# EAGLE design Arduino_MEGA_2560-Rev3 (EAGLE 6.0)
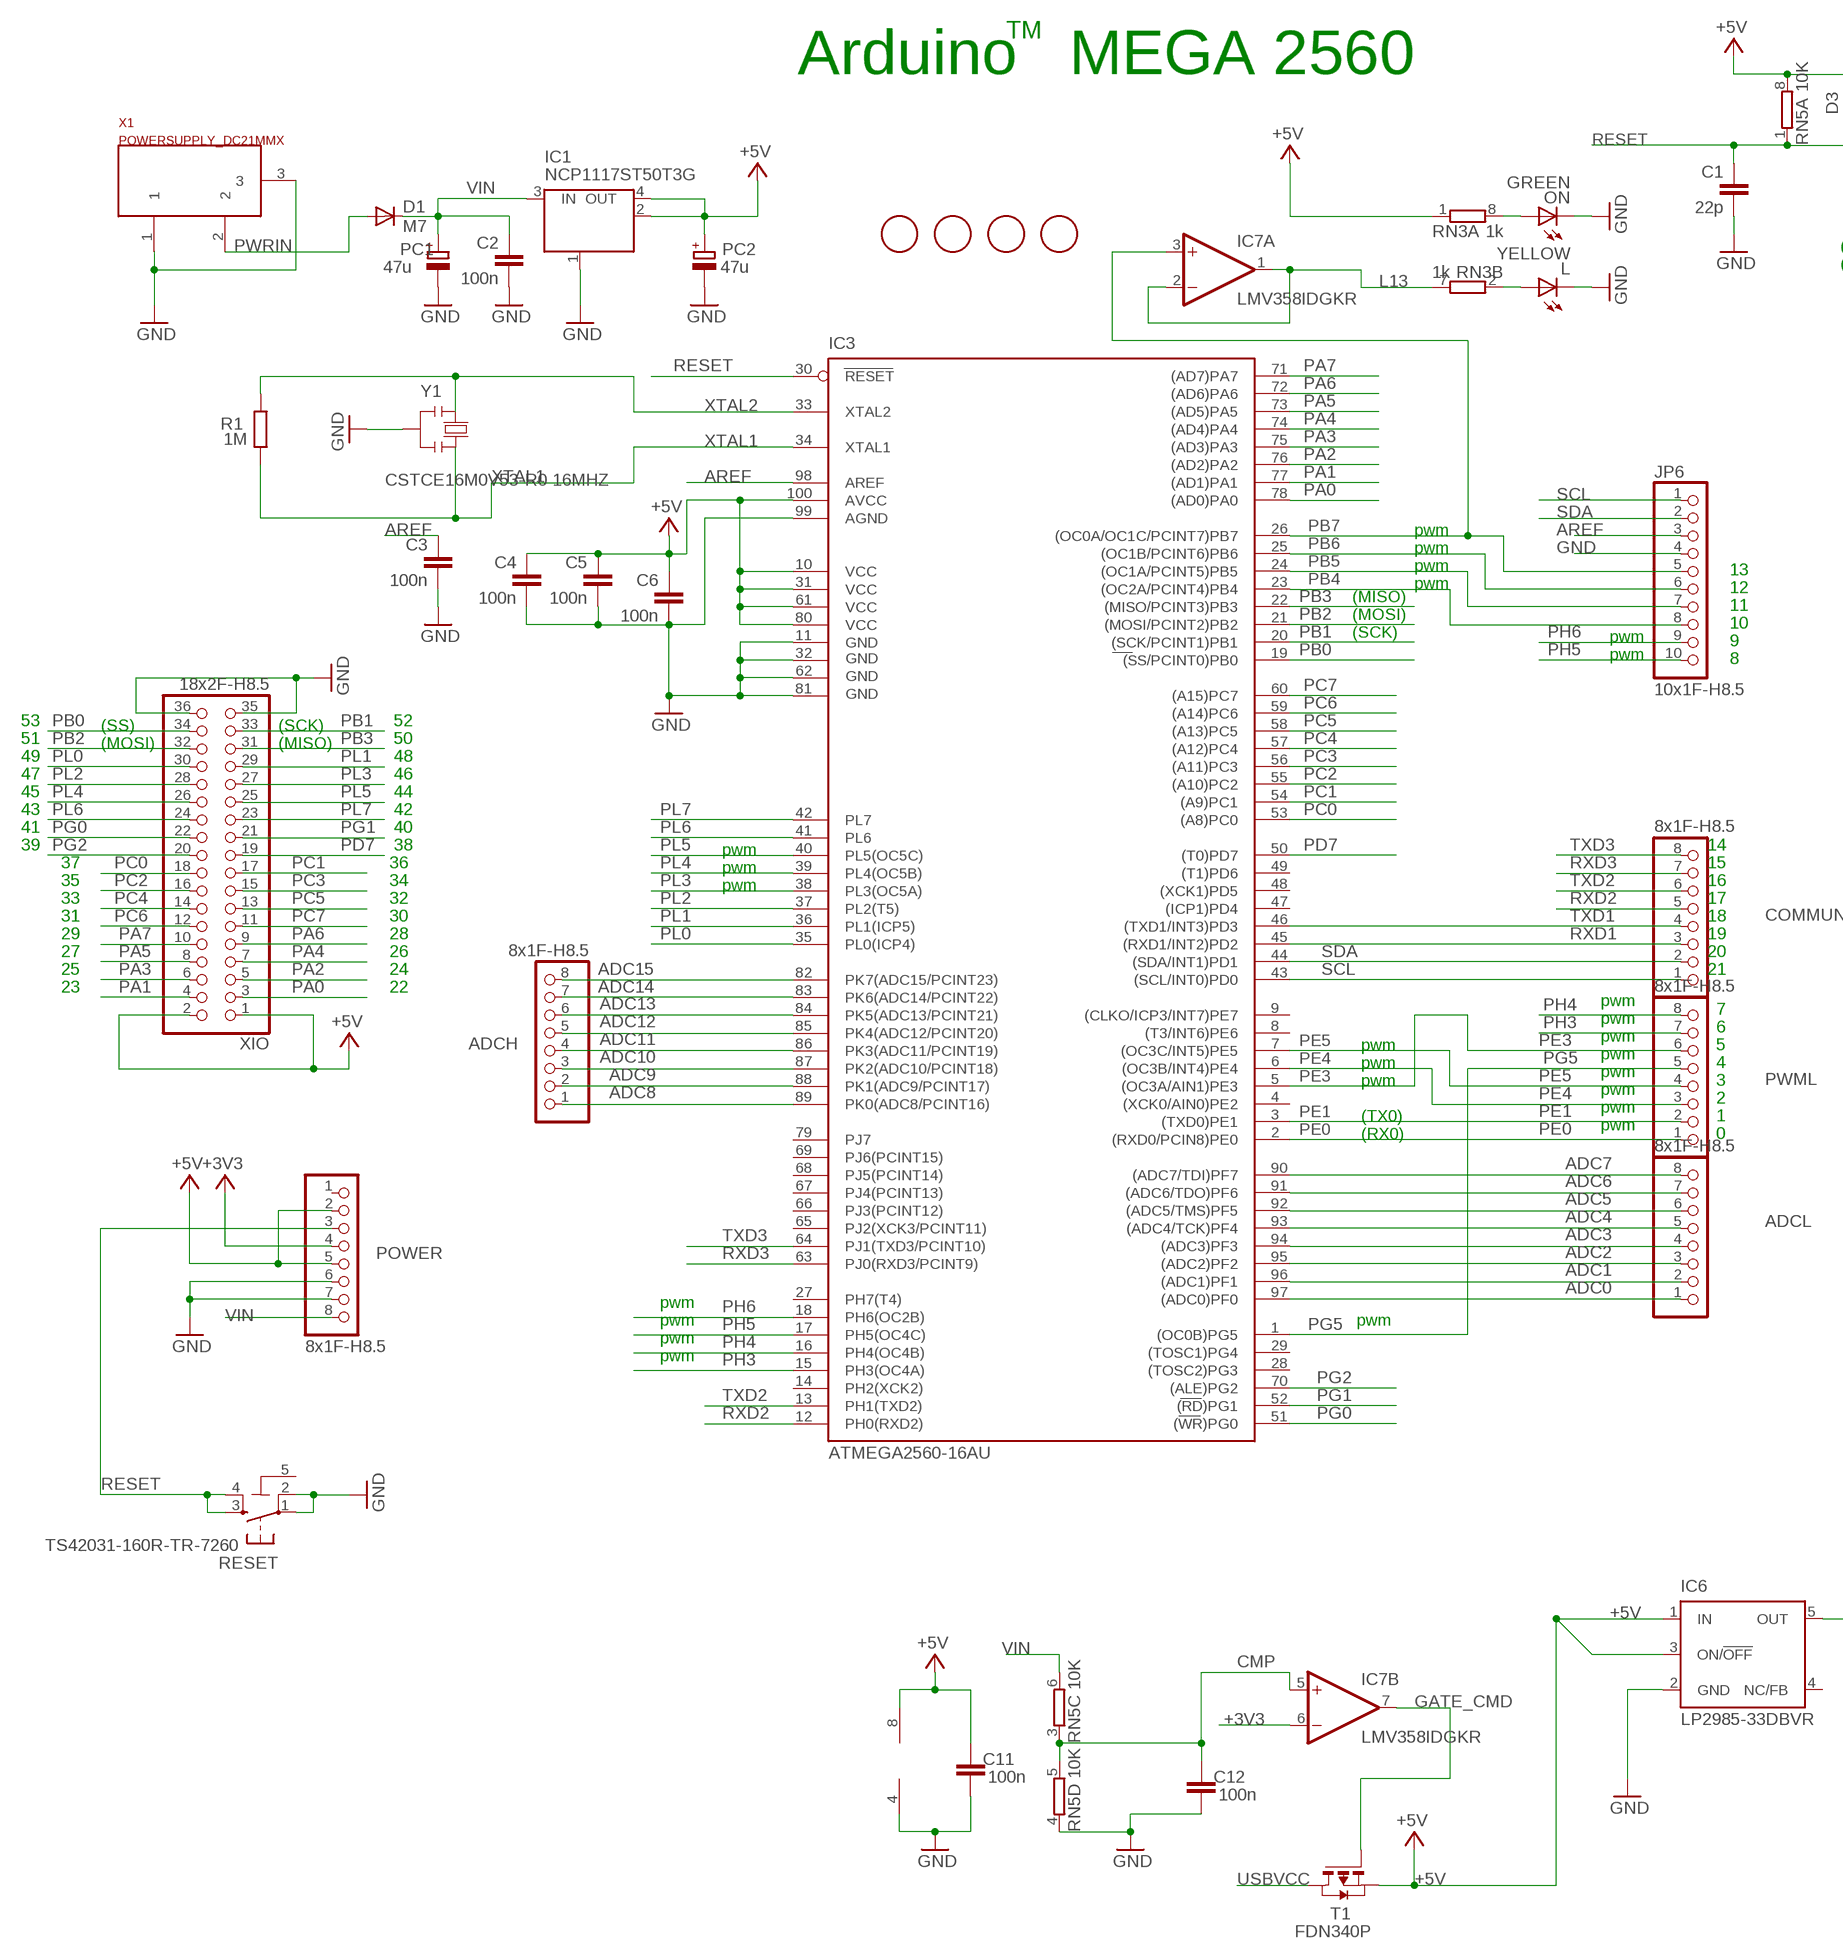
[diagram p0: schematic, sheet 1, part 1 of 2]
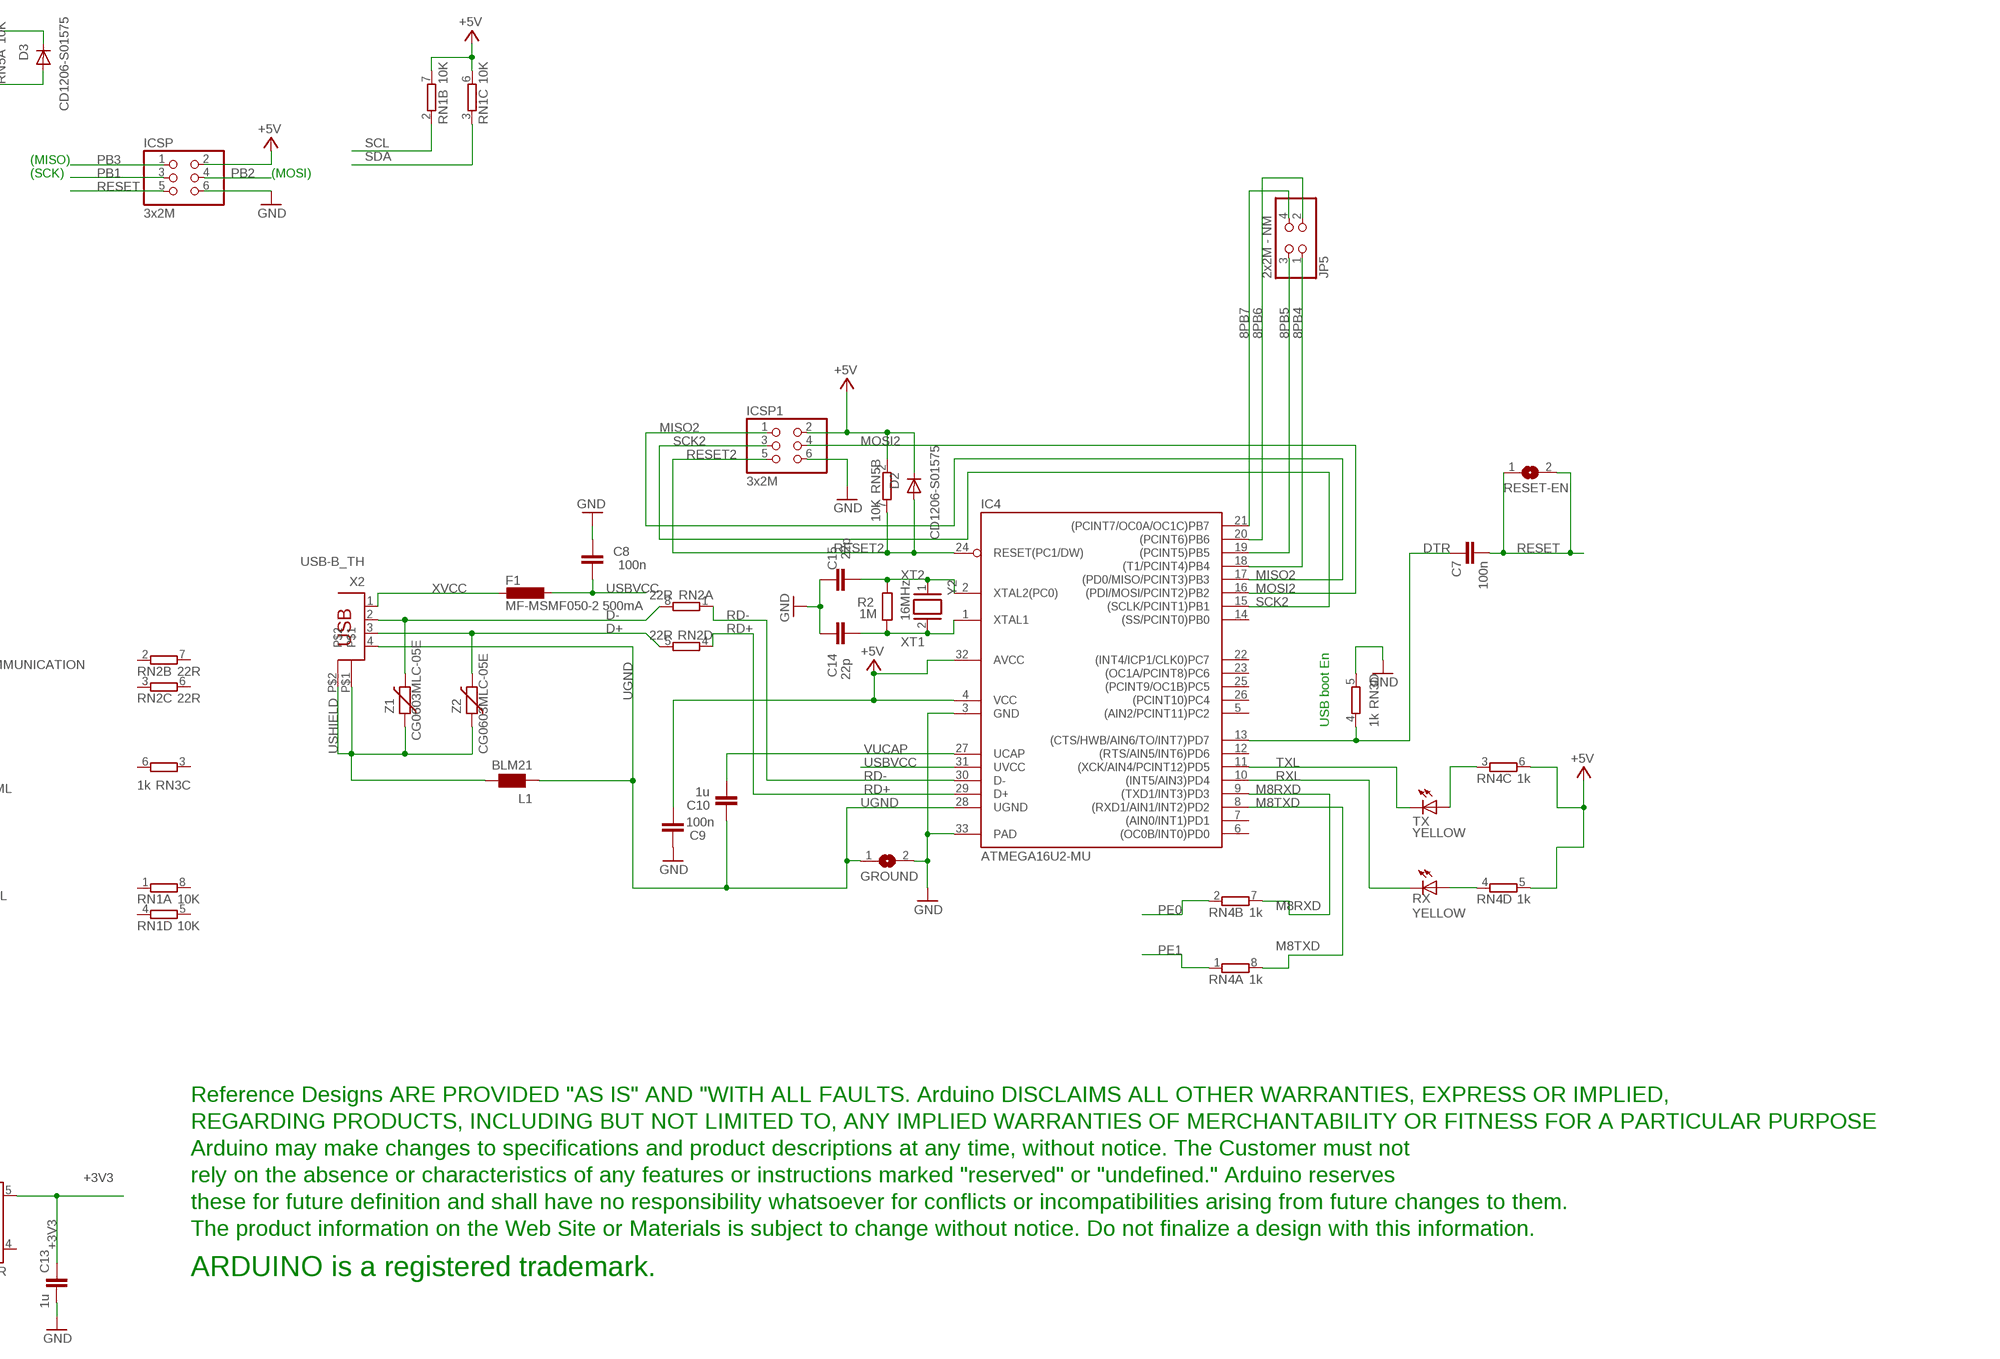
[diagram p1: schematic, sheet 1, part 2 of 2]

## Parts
ADCH  8x1F-H8.5  PINHD-1X8  [1X08]
ADCL  8x1F-H8.5  PINHD-1X8  [1X08]
C1  22p  C-EU0603-RND  [C0603-ROUND]
C2  100n  C-EU0603-RND  [C0603-ROUND]
C3  100n  C-EU0603-RND  [C0603-ROUND]
C4  100n  C-EU0603-RND  [C0603-ROUND]
C5  100n  C-EU0603-RND  [C0603-ROUND]
C6  100n  C-EU0603-RND  [C0603-ROUND]
C7  100n  C-EU0603-RND  [C0603-ROUND]
C8  100n  C-EU0603-RND  [C0603-ROUND]
C9  100n  C-EU0603-RND  [C0603-ROUND]
C10  1u  C-EU0603-RND  [C0603-ROUND]
C11  100n  C-EU0603-RND  [C0603-ROUND]
C12  100n  C-EU0603-RND  [C0603-ROUND]
C13  1u  C-EU0603-RND  [C0603-ROUND]
C14  22p  C-EU0603-RND  [C0603-ROUND]
C15  22p  C-EU0603-RND  [C0603-ROUND]
COMMUNICATION  8x1F-H8.5  PINHD-1X8  [1X08]
D1  M7  DIODE-SMB  [SMB]
D2  CD1206-S01575  DIODE-MINIMELF  [MINIMELF]
D3  CD1206-S01575  DIODE-MINIMELF  [MINIMELF]
F1  MF-MSMF050-2 500mA  L-EUL1812  [L1812]
FD1  FIDUCIALMOUNT  [FIDUCIA-MOUNT]
FD2  FIDUCIALMOUNT  [FIDUCIA-MOUNT]
FD3  FIDUCIALMOUNT  [FIDUCIA-MOUNT]
FD4  FIDUCIALMOUNT  [FIDUCIA-MOUNT]
GROUND  SJ  [SJ]
IC1  NCP1117ST50T3G  MC33269ST-3.3T3  [SOT223]
IC3  ATMEGA2560-16AU  ATMEGA25602560-16AU  [TQFP100]
IC4  ATMEGA16U2-MU  [MLF32]
IC6  LP2985-33DBVR  LP2985-XXDBVR33  [SOT23-DBV]
IC7  LMV358IDGKR  LMV358MMX  [MSOP08]
ICSP  3x2M  PINHD-2X3  [2X03]
ICSP1  3x2M  PINHD-2X3  [2X03]
JP5  2x2M - NM  PINHD-2X2  [2X02]
JP6  10x1F-H8.5  PINHD-1X10_ARD  [1X10]
L  YELLOW  LEDCHIP-LED0805  [CHIP-LED0805]
L1  BLM21  WE-CBF_0805  [0805]
ON  GREEN  LEDCHIP-LED0805  [CHIP-LED0805]
PC1  47u  CPOL-EUD  [PANASONIC_D]
PC2  47u  CPOL-EUD  [PANASONIC_D]
POWER  8x1F-H8.5  PINHD-1X8  [1X08]
PWML  8x1F-H8.5  PINHD-1X8  [1X08]
R1  1M  R-EU_R0603  [R0603-ROUND]
R2  1M  R-EU_R0603  [R0603-ROUND]
RESET  TS42031-160R-TR-7260  TS42  [TS42]
RESET-EN  SJ  [SJ]
RN1  10K  4R-NCAT16  [CAT16]
RN2  22R  4R-NCAY16  [CAY16]
RN3  1k  4R-NCAY16  [CAY16]
RN4  1k  4R-NCAY16  [CAY16]
RN5  10K  4R-NCAT16  [CAT16]
RX  YELLOW  LEDCHIP-LED0805  [CHIP-LED0805]
T1  FDN340P  PMOSSOT23  [SOT-23]
TX  YELLOW  LEDCHIP-LED0805  [CHIP-LED0805]
U$1  DISCLAIMER  [DISCLAIMER]
X1  POWERSUPPLY_DC21MMX  [POWERSUPPLY_DC-21MM]
X2  USB-B_TH  PN61729  [PN61729]
XIO  18x2F-H8.5  PINHD-2X18  [2X18]
Y1  CSTCE16M0V53-R0 16MHZ  RESONATORMU  [RESONATOR]
Y2  16MHz  XTAL/S  [QS]
Z1  CG0603MLC-05E  VARISTORCN0603  [CT/CN0603]
Z2  CG0603MLC-05E  VARISTORCN0603  [CT/CN0603]

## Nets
8PB4: IC4.18((T1/PCINT4)PB4) JP5.1
8PB5: IC4.19((PCINT5)PB5) JP5.3
8PB6: IC4.20((PCINT6)PB6) JP5.2
8PB7: IC4.21((PCINT7/OC0A/OC1C)PB7) JP5.4
+3V3 [power]: C13.2 IC6.5(OUT) IC7.6(B:-IN) POWER.4
+5V [power usb]: C4.1 C5.1 C6.1 C9.1 C11.2 D2.C D3.C IC1.2(OUT) IC1.4(OUT) IC3.10(VCC) IC3.31(VCC1) IC3.61(VCC2) IC3.80(VCC3) IC3.100(AVCC) IC4.4(VCC) IC4.32(AVCC) IC6.1(IN) IC6.3(ON/!OFF) IC7.8(P:V+) ICSP1.2 ICSP.2 PC2.+ POWER.2 POWER.5 RN1.6 RN1.7 RN3.1 RN4.5 RN4.6 RN5.2 RN5.8 T1.2(S) XIO.1 XIO.2
ADC0: ADCL.1 IC3.97((ADC0)PF0)
ADC1: ADCL.2 IC3.96((ADC1)PF1)
ADC2: ADCL.3 IC3.95((ADC2)PF2)
ADC3: ADCL.4 IC3.94((ADC3)PF3)
ADC4: ADCL.5 IC3.93((ADC4/TCK)PF4)
ADC5: ADCL.6 IC3.92((ADC5/TMS)PF5)
ADC6: ADCL.7 IC3.91((ADC6/TDO)PF6)
ADC7: ADCL.8 IC3.90((ADC7/TDI)PF7)
ADC8: ADCH.1 IC3.89(PK0(ADC8/PCINT16))
ADC9: ADCH.2 IC3.88(PK1(ADC9/PCINT17))
ADC10: ADCH.3 IC3.87(PK2(ADC10/PCINT18))
ADC11: ADCH.4 IC3.86(PK3(ADC11/PCINT19))
ADC12: ADCH.5 IC3.85(PK4(ADC12/PCINT20))
ADC13: ADCH.6 IC3.84(PK5(ADC13/PCINT21))
ADC14: ADCH.7 IC3.83(PK6(ADC14/PCINT22))
ADC15: ADCH.8 IC3.82(PK7(ADC15/PCINT23))
AREF: C3.1 IC3.98(AREF) JP6.3
CMP: C12.2 IC7.5(B:+IN) RN5.3 RN5.5
D+: RN2.5 X2.3 Z2.2
D-: RN2.8 X2.2 Z1.2
DTR: C7.1 IC4.13((CTS/HWB/AIN6/TO/INT7)PD7) RN3.4
GATE_CMD: IC7.7(B:OUT) T1.3(G)
GND [gnd]: C1.2 C2.2 C3.2 C4.2 C5.2 C6.2 C8.2 C9.2 C11.1 C12.1 C13.1 C14.2 C15.2 GROUND.2 IC1.1(GND/ADJ) IC3.11(GND) IC3.32(GND1) IC3.62(GND2) IC3.81(GND3) IC3.99(AGND) IC4.3(GND) IC4.33(PAD) IC6.2(GND) IC7.4(P:V-) ICSP1.6 ICSP.6 JP6.4 L.C ON.C PC1.- PC2.- POWER.6 POWER.7 RESET.1 RESET.2 RN3.5 RN5.4 X1.1 X1.3 XIO.35 XIO.36 Y1.2
L13: IC7.1(A:OUT) IC7.2(A:-IN) RN3.7
M8RXD: IC4.9((TXD1/INT3)PD3) RN4.7
M8TXD: IC4.8((RXD1/AIN1/INT2)PD2) RN4.8
MISO2: IC4.17((PD0/MISO/PCINT3)PB3) ICSP1.1
MOSI2: IC4.16((PDI/MOSI/PCINT2)PB2) ICSP1.4
N$2: L.A RN3.2
N$3: ON.A RN3.8
N$54: RN4.4 RX.A
N$55: RN4.3 TX.A
PA0: IC3.78((AD0)PA0) XIO.3
PA1: IC3.77((AD1)PA1) XIO.4
PA2: IC3.76((AD2)PA2) XIO.5
PA3: IC3.75((AD3)PA3) XIO.6
PA4: IC3.74((AD4)PA4) XIO.7
PA5: IC3.73((AD5)PA5) XIO.8
PA6: IC3.72((AD6)PA6) XIO.9
PA7: IC3.71((AD7)PA7) XIO.10
PB0: IC3.19((SS/PCINT0)PB0) XIO.34
PB1: IC3.20((SCK/PCINT1)PB1) ICSP.3 XIO.33
PB2: IC3.21((MOSI/PCINT2)PB2) ICSP.4 XIO.32
PB3: IC3.22((MISO/PCINT3)PB3) ICSP.1 XIO.31
PB4: IC3.23((OC2A/PCINT4)PB4) JP6.8
PB5: IC3.24((OC1A/PCINT5)PB5) JP6.7
PB6: IC3.25((OC1B/PCINT6)PB6) JP6.6
PB7: IC3.26((OC0A/OC1C/PCINT7)PB7) IC7.3(A:+IN) JP6.5
PC0: IC3.53((A8)PC0) XIO.18
PC1: IC3.54((A9)PC1) XIO.17
PC2: IC3.55((A10)PC2) XIO.16
PC3: IC3.56((A11)PC3) XIO.15
PC4: IC3.57((A12)PC4) XIO.14
PC5: IC3.58((A13)PC5) XIO.13
PC6: IC3.59((A14)PC6) XIO.12
PC7: IC3.60((A15)PC7) XIO.11
PD7: IC3.50((T0)PD7) XIO.19
PE0: IC3.2((RXD0/PCIN8)PE0) PWML.1 RN4.2
PE1: IC3.3((TXD0)PE1) PWML.2 RN4.1
PE3: IC3.5((OC3A/AIN1)PE3) PWML.6
PE4: IC3.6((OC3B/INT4)PE4) PWML.3
PE5: IC3.7((OC3C/INT5)PE5) PWML.4
PG0: IC3.51((WR)PG0) XIO.22
PG1: IC3.52((RD)PG1) XIO.21
PG2: IC3.70((ALE)PG2) XIO.20
PG5: IC3.1((OC0B)PG5) PWML.5
PH3: IC3.15(PH3(OC4A)) PWML.7
PH4: IC3.16(PH4(OC4B)) PWML.8
PH5: IC3.17(PH5(OC4C)) JP6.10
PH6: IC3.18(PH6(OC2B)) JP6.9
PL0: IC3.35(PL0(ICP4)) XIO.30
PL1: IC3.36(PL1(ICP5)) XIO.29
PL2: IC3.37(PL2(T5)) XIO.28
PL3: IC3.38(PL3(OC5A)) XIO.27
PL4: IC3.39(PL4(OC5B)) XIO.26
PL5: IC3.40(PL5(OC5C)) XIO.25
PL6: IC3.41(PL6) XIO.24
PL7: IC3.42(PL7) XIO.23
PWRIN [power]: D1.A X1.2
RD+: IC4.29(D+) RN2.4
RD-: IC4.30(D-) RN2.1
RESET: C1.1 C7.2 D3.A IC3.30(RESET) ICSP.5 POWER.3 RESET-EN.1 RESET-EN.2 RESET.3 RESET.4 RN5.1
RESET2: D2.A IC4.24(RESET(PC1/DW)) ICSP1.5 RN5.7
RXD1: COMMUNICATION.3 IC3.45((RXD1/INT2)PD2)
RXD2: COMMUNICATION.5 IC3.12(PH0(RXD2))
RXD3: COMMUNICATION.7 IC3.63(PJ0(RXD3/PCINT9))
RXL: IC4.10((INT5/AIN3)PD4) RX.C
SCK2: IC4.15((SCLK/PCINT1)PB1) ICSP1.3
SCL: COMMUNICATION.1 IC3.43((SCL/INT0)PD0) JP6.1 RN1.2
SDA: COMMUNICATION.2 IC3.44((SDA/INT1)PD1) JP6.2 RN1.3
TXD1: COMMUNICATION.4 IC3.46((TXD1/INT3)PD3)
TXD2: COMMUNICATION.6 IC3.13(PH1(TXD2))
TXD3: COMMUNICATION.8 IC3.64(PJ1(TXD3/PCINT10))
TXL: IC4.11((XCK/AIN4/PCINT12)PD5) TX.C
UGND [gnd]: C10.2 GROUND.1 IC4.28(UGND) L1.1 X2.4
USBVCC [power usb]: C8.1 F1.1 IC4.31(UVCC) T1.1(D)
USHIELD [gnd]: L1.2 X2.P$1 X2.P$2 Z1.1 Z2.1
VIN [power]: C2.1 D1.C IC1.3(IN) PC1.+ POWER.8 RN5.6
VUCAP: C10.1 IC4.27(UCAP)
XT1: C14.1 IC4.1(XTAL1) R2.1 Y2.2
XT2: C15.1 IC4.2(XTAL2(PC0)) R2.2 Y2.1
XTAL1: IC3.34(XTAL1) R1.1 Y1.3
XTAL2: IC3.33(XTAL2) R1.2 Y1.1
XVCC [power usb]: F1.2 X2.1
Unconnected: IC3.4((XCK0/AIN0)PE2) IC3.8((T3/INT6)PE6) IC3.9((CLKO/ICP3/INT7)PE7) IC3.14(PH2(XCK2)) IC3.27(PH7(T4)) IC3.28((TOSC2)PG3) IC3.29((TOSC1)PG4) IC3.47((ICP1)PD4) IC3.48((XCK1)PD5) IC3.49((T1)PD6) IC3.65(PJ2(XCK3/PCINT11)) IC3.66(PJ3(PCINT12)) IC3.67(PJ4(PCINT13)) IC3.68(PJ5(PCINT14)) IC3.69(PJ6(PCINT15)) IC3.79(PJ7) IC4.5((AIN2/PCINT11)PC2) IC4.6((OC0B/INT0)PD0) IC4.7((AIN0/INT1)PD1) IC4.12((RTS/AIN5/INT6)PD6) IC4.14((SS/PCINT0)PB0) IC4.22((INT4/ICP1/CLK0)PC7) IC4.23((OC1A/PCINT8)PC6) IC4.25((PCINT9/OC1B)PC5) IC4.26((PCINT10)PC4) IC6.4(NC/FB) POWER.1 RN1.1 RN1.4 RN1.5 RN1.8 RN2.2 RN2.3 RN2.6 RN2.7 RN3.3 RN3.6

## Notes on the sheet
- TM
- Arduino   MEGA 2560
- (MISO)
- (SCK) | (MOSI)
- pwm
- pwm
- pwm | 13
- pwm | 12
- (MISO)
- 11
- (MOSI)
- 10
- (SCK) | pwm
- 9
- pwm | 8
- 53 | (SS) | (SCK) | 52
- 51 | (MOSI) | (MISO) | 50
- 49 | 48
- 47 | 46
- 45 | 44
- 43 | 42
- 41 | 40
- 39 | 38 | pwm | 14
- 37 | 36 | pwm | 15
- 35 | 34 | pwm | 16
- 33 | 32 | 17
- 31 | 30 | 18
- 29 | 28 | 19
- 27 | 26 | 20
- 25 | 24 | 21
- 23 | 22 | USB boot En
- pwm
- 7
- pwm
- 6
- pwm
- pwm | 5
- pwm
- pwm | 4
- pwm
- pwm | 3
- pwm
- 2
- pwm
- (TX0) | 1
- pwm
- (RX0) | 0
- pwm
- pwm | pwm
- pwm
- pwm

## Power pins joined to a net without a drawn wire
5-GND: RESET.5(5-GND)

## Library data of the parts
ADCH ADCL COMMUNICATION POWER PWML = SmartPrj:PINHD-1X8: PIN HEADER
C1-C15 = SmartPrj:C-EU: CAPACITOR, European symbol
D1-D3 = diode:DIODE-: DIODE
F1 = rcl:L-EU: INDUCTOR, European symbol
FD1-FD4 = SmartPrj:FIDUCIALMOUNT
GROUND RESET-EN = jumper:SJ: SMD solder JUMPER
IC1 = linear:MC33269ST*: Adjustable Output Low Dropout Voltage Regulator 800 mA Source: http://www.onsemi.com/pub/Collateral/MC33269-D.PDF
IC3 = SmartPrj:ATMEGA2560: MICROCONTROLLER 64/128/256 Kbytes FLASH 4 Kbytes EEPROM 8 Kbytes SRAM 86 General Purpose I/O pins 12-channels16-bit PWM 4 x Serial USARTs 16-channels 10-bit A/D
IC4 = SmartPrj:ATMEGA16U2-
IC6 = SmartPrj:LP2985-XXDBVR: ULTRALOW-POWER 50-mA LOW-DROPOUT LINEAR REGULATORS 50-mA Low-Dropout Regulator Source: http://focus.ti.com/lit/ds/symlink/tps77001.pdf
IC7 = linear:LMV358?*: Dual General Purpose, Low Voltage, Rail-to-Rail Output Operational Amplifiers Source: http://www.national.com/mpf/LM/LMV321.html http://www.national.com/dt/lmv_qual.pdf
ICSP ICSP1 = SmartPrj:PINHD-2X3: PIN HEADER
JP5 = SmartPrj:PINHD-2X2: PIN HEADER
JP6 = SmartPrj:PINHD-1X10_ARD: PIN HEADER
L ON RX TX = led:LED: LED
L1 = wuerth-elektronik:WE-CBF: SMD EMI Suppression Ferrite Beads
PC1 PC2 = rcl:CPOL-EU: POLARIZED CAPACITOR, European symbol
R1 R2 = SmartPrj:R-EU_: RESISTOR, European symbol
RESET = SmartPrj:TS42: TS42 Dongnan Electronics Tact switch VDC 12V - 50mA
RN1-RN5 = resistor-dil:4R-N: Array Chip Resistor Source: RS Component / Phycomp
T1 = zetex:PMOSSOT23: MOS FET
U$1 = SmartPrj:DISCLAIMER
X1 = SmartPrj:POWERSUPPLY_DC21MM
X2 = SmartPrj:PN61729: BERG USB connector
XIO = SmartPrj:PINHD-2X18: PIN HEADER
Y1 = SmartPrj:RESONATOR
Y2 = SmartPrj:XTAL/S: CRYSTAL
Z1 Z2 = varistor:VARISTOR: VARISTOR

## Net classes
0 default: width 0.203 mm, drill 0.406 mm, clearance 0.203 mm
1 power: width 0.61 mm, drill 0.406 mm, clearance 0.203 mm
2 gnd: width 0.305 mm, drill 0.406 mm, clearance 0.203 mm
3 power usb: width 0.508 mm, drill 0.406 mm, clearance 0.203 mm

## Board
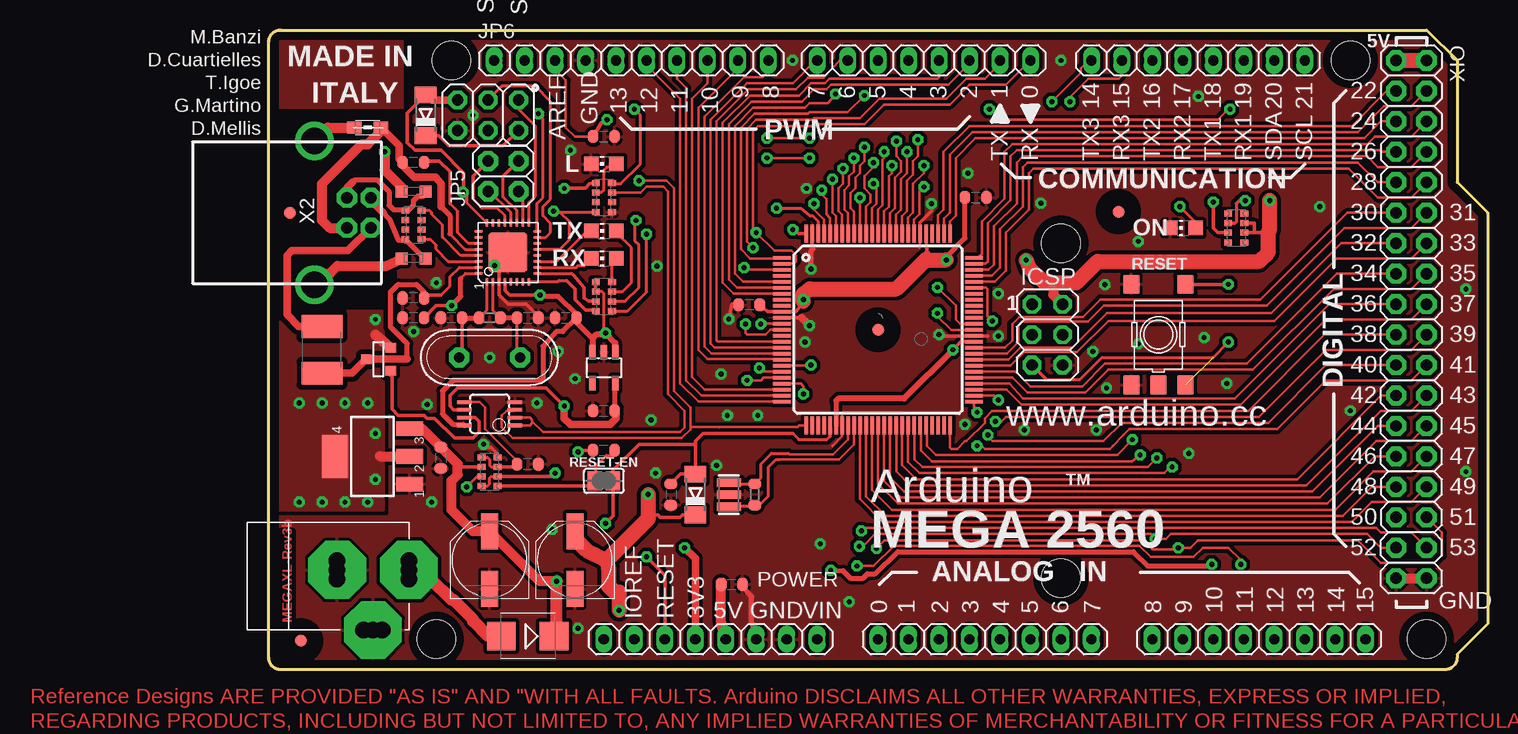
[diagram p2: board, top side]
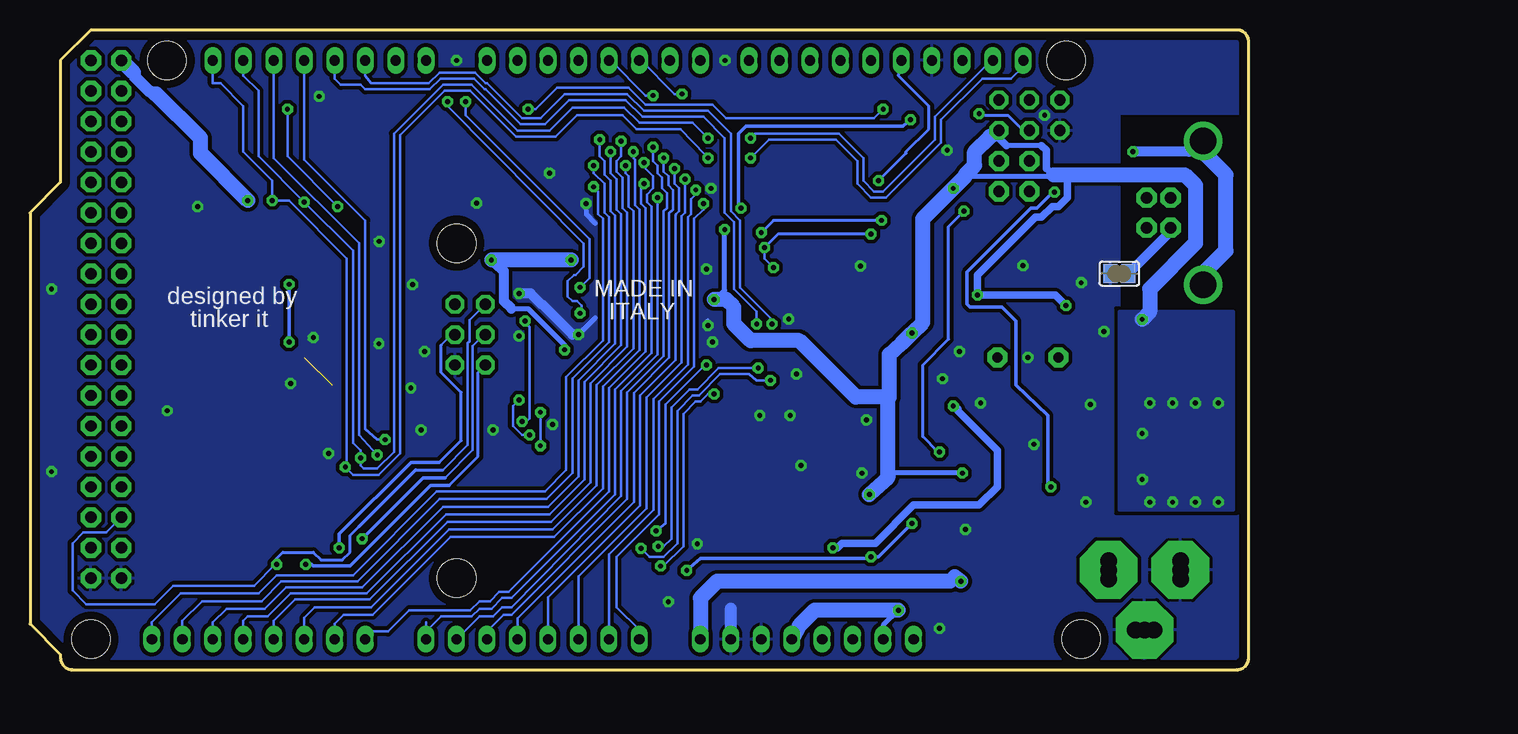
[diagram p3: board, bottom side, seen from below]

Size 101.6 x 53.34 mm. Coordinates in mm from the lower left corner, seen from the top.
Outline: 96.52,53.34 99.06,50.8 99.06,40.64 101.6,38.1 101.6,3.81 99.06,1.27 99.06,1 arc-90 98.06,0 1,0 arc-90 0,1 0,52.34 arc-90 1,53.34 96.52,53.34
Copper layers (1*16): Top 0.035mm / dielectric 1.5mm / Bottom 0.035mm
Design rules: minimum track width 8mil, minimum drill 16mil, track to track 7mil, track to pad 7mil, pad to pad 8mil, via to via 10mil, smd to smd 7mil, copper to edge 27mil, drill to drill 12mil, minimum pad ring 10mil, minimum via ring 10mil, stop-mask expansion 2mil, vias tented up to drill 24mil, thermal gap 10mil
Holes 3.2 mm at 96.52,2.54 15.24,50.8 90.17,50.8 13.97,2.54 66.04,35.56 66.04,7.62

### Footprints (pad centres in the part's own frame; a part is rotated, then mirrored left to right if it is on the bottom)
1X08 = drill 0.85 pad 1.422 long: 1 -8.89,0; 2 -6.35,0; 3 -3.81,0; 4 -1.27,0; 5 1.27,0; 6 3.81,0; 7 6.35,0; 8 8.89,0
C0603-ROUND = smd 0.898 x 1.1: 1 -0.889,0; 2 0.889,0
SMB = smd 2.4 x 2.4: A 2.2,0; C -2.2,0
MINIMELF = smd 1.4 x 1.8: A 1.7,0; C -1.7,0
L1812 = smd 1.9 x 3.4: 1 -1.95,0; 2 1.95,0
FIDUCIA-MOUNT = smd 1.016 x 1.016: P$1 0,0
SJ = smd 1.168 x 1.6: 1 -0.762,0; 2 0.762,0
SOT223 = smd 1.219 x 2.235: 1 -2.311,-3.099; 2 0,-3.099; 3 2.311,-3.099 | smd 3.6 x 2.2: 4 0,3.099
TQFP100 = smd 1.5 x 0.3: 1 -8,6; 2 -8,5.5; 3 -8,5; 4 -8,4.5; 5 -8,4; 6 -8,3.5; 7 -8,3; 8 -8,2.5; 9 -8,2; 10 -8,1.5; 11 -8,1; 12 -8,0.5; 13 -8,0; 14 -8,-0.5; 15 -8,-1; 16 -8,-1.5; 17 -8,-2; 18 -8,-2.5; 19 -8,-3; 20 -8,-3.5; 21 -8,-4; 22 -8,-4.5; 23 -8,-5; 24 -8,-5.5; 25 -8,-6; 51 8,-6; 52 8,-5.5; 53 8,-5; 54 8,-4.5; 55 8,-4; 56 8,-3.5; 57 8,-3; 58 8,-2.5; 59 8,-2; 60 8,-1.5; 61 8,-1; 62 8,-0.5; 63 8,0; 64 8,0.5; 65 8,1; 66 8,1.5; 67 8,2; 68 8,2.5; 69 8,3; 70 8,3.5; 71 8,4; 72 8,4.5; 73 8,5; 74 8,5.5; 75 8,6 | smd 0.3 x 1.5: 26 -6,-8; 27 -5.5,-8; 28 -5,-8; 29 -4.5,-8; 30 -4,-8; 31 -3.5,-8; 32 -3,-8; 33 -2.5,-8; 34 -2,-8; 35 -1.5,-8; 36 -1,-8; 37 -0.5,-8; 38 0,-8; 39 0.5,-8; 40 1,-8; 41 1.5,-8; 42 2,-8; 43 2.5,-8; 44 3,-8; 45 3.5,-8; 46 4,-8; 47 4.5,-8; 48 5,-8; 49 5.5,-8; 50 6,-8; 76 6,8; 77 5.5,8; 78 5,8; 79 4.5,8; 80 4,8; 81 3.5,8; 82 3,8; 83 2.5,8; 84 2,8; 85 1.5,8; 86 1,8; 87 0.5,8; 88 0,8; 89 -0.5,8; 90 -1,8; 91 -1.5,8; 92 -2,8; 93 -2.5,8; 94 -3,8; 95 -3.5,8; 96 -4,8; 97 -4.5,8; 98 -5,8; 99 -5.5,8; 100 -6,8
MLF32 = smd 0.7 x 0.28: 1 -2.45,1.75; 2 -2.45,1.25; 3 -2.45,0.75; 4 -2.45,0.25; 5 -2.45,-0.25; 6 -2.45,-0.75; 7 -2.45,-1.25; 8 -2.45,-1.75; 17 2.45,-1.75; 18 2.45,-1.25; 19 2.45,-0.75; 20 2.45,-0.25; 21 2.45,0.25; 22 2.45,0.75; 23 2.45,1.25; 24 2.45,1.75 | smd 0.28 x 0.7: 9 -1.75,-2.45; 10 -1.25,-2.45; 11 -0.75,-2.45; 12 -0.25,-2.45; 13 0.25,-2.45; 14 0.75,-2.45; 15 1.25,-2.45; 16 1.75,-2.45; 25 1.75,2.45; 26 1.25,2.45; 27 0.75,2.45; 28 0.25,2.45; 29 -0.25,2.45; 30 -0.75,2.45; 31 -1.25,2.45; 32 -1.75,2.45 | smd 3.254 x 3.254: 33 0,0
SOT23-DBV = smd 0.55 x 1.2: 1 -0.95,-1.3; 2 0,-1.3; 3 0.95,-1.3; 4 0.95,1.3; 5 -0.95,1.3
MSOP08 = smd 0.3 x 1.2: 1 -0.976,-2.113; 2 -0.326,-2.113; 3 0.324,-2.113; 4 0.974,-2.113; 5 0.974,2.112; 6 0.324,2.112; 7 -0.326,2.112; 8 -0.976,2.112
2X03 = drill 0.95 pad 1.55 octagon: 1 -2.54,-1.27; 2 -2.54,1.27; 3 0,-1.27; 4 0,1.27; 5 2.54,-1.27; 6 2.54,1.27
2X02 = drill 0.95 pad 1.676 octagon: 1 -1.27,-1.27; 2 -1.27,1.27; 3 1.27,-1.27; 4 1.27,1.27
1X10 = drill 0.85 pad 1.422 long: 1 -11.43,0; 2 -8.89,0; 3 -6.35,0; 4 -3.81,0; 5 -1.27,0; 6 1.27,0; 7 3.81,0; 8 6.35,0; 9 8.89,0; 10 11.43,0
CHIP-LED0805 = smd 1.2 x 1.2: A 0,-1.05; C 0,1.05
0805 = smd 1.2 x 1: 1 -1.1,0; 2 1.1,0
PANASONIC_D = smd 3 x 1.4: + 2.4,0; - -2.4,0
R0603-ROUND = smd 0.898 x 1.1: 1 -0.889,0; 2 0.889,0
TS42 = smd 1.6 x 1.4: 1 -4.2,2.25; 2 4.2,2.25; 3 -4.2,-2.25; 4 4.2,-2.25; 5 -4.2,0
CAT16 = smd 0.5 x 0.65: 1 -1.2,-0.675; 2 -0.4,-0.675; 3 0.4,-0.675; 4 1.2,-0.675; 5 1.2,0.675; 6 0.4,0.675; 7 -0.4,0.675; 8 -1.2,0.675
CAY16 = smd 0.5 x 0.65: 1 -1.2,-0.675; 2 -0.4,-0.675; 3 0.4,-0.675; 4 1.2,-0.675; 5 1.2,0.675; 6 0.4,0.675; 7 -0.4,0.675; 8 -1.2,0.675
SOT-23 = smd 0.787 x 0.889: 1 0.025,-1.016; 2 -0.94,1.016; 3 0.991,1.016
POWERSUPPLY_DC-21MM = drill 1.4 pad 4.826 octagon: 1 -5.08,-3.353; 2 -0.076,-6.35; 3 -0.076,-0.356 | drill 1.4: 4 -5.08,-4.115; 5 -5.08,-2.591; 6 -0.838,-0.356; 7 0.686,-0.356; 8 -0.838,-6.35; 9 0.686,-6.35
PN61729 = drill 0.95 pad 1.676 octagon: 1 1.25,4.71; 2 -1.25,4.71; 3 -1.25,2.71; 4 1.25,2.71 | drill 2.2: P$1 -6,0; P$2 6,0
2X18 = drill 0.95 pad 1.676 octagon: 1 -21.59,-1.27; 2 -21.59,1.27; 3 -19.05,-1.27; 4 -19.05,1.27; 5 -16.51,-1.27; 6 -16.51,1.27; 7 -13.97,-1.27; 8 -13.97,1.27; 9 -11.43,-1.27; 10 -11.43,1.27; 11 -8.89,-1.27; 12 -8.89,1.27; 13 -6.35,-1.27; 14 -6.35,1.27; 15 -3.81,-1.27; 16 -3.81,1.27; 17 -1.27,-1.27; 18 -1.27,1.27; 19 1.27,-1.27; 20 1.27,1.27; 21 3.81,-1.27; 22 3.81,1.27; 23 6.35,-1.27; 24 6.35,1.27; 25 8.89,-1.27; 26 8.89,1.27; 27 11.43,-1.27; 28 11.43,1.27; 29 13.97,-1.27; 30 13.97,1.27; 31 16.51,-1.27; 32 16.51,1.27; 33 19.05,-1.27; 34 19.05,1.27; 35 21.59,-1.27; 36 21.59,1.27
RESONATOR = smd 0.7 x 2: 1 -1,0; 2 0,0; 3 1,0
QS = drill 0.85 pad 1.676 octagon: 1 -2.54,0; 2 2.54,0
CT/CN0603 = smd 1 x 1: 1 -1,0; 2 1,0

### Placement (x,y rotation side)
ADCH  82.55,2.54 0 top
ADCL  59.69,2.54 0 top
C1  33.53,14.61 270 top
C2  14.35,17.65 270 top
C3  27.94,44.45 0 top
C4  38.61,7.11 0 top
C5  58.93,39.37 0 top
C6  40.05,30.42 180 top
C7  27.94,18.29 0 top
C8  12.06,30.99 180 top
C9  12.06,29.34 180 top
C10  12.06,42.29 180 top
C11  24.77,29.34 0 top
C12  21.59,17.14 180 top
C13  27.94,21.59 0 top
C14  15.24,29.34 180 top
C15  21.59,29.34 0 top
COMMUNICATION  77.47,50.8 180 top
D1  21.59,2.79 180 top
D2  13.08,46.23 90 top
D3  35.56,14.61 90 top
F1  4.45,26.67 90 top
FD1  70.84,38.19 0 top
FD2  2.67,2.41 0 top
FD3  1.78,38.1 0 top
FD4  50.8,28.35 0 top
GROUND  10.79,33.02 180 bottom
IC1  8.64,17.78 90 top
IC3  50.8,28.35 0 top
IC4  19.94,34.8 90 top
IC6  27.94,25.17 180 top
IC7  18.41,21.34 90 top
ICSP  64.9,27.94 270 top
ICSP1  18.29,46.23 180 top
JP5  19.56,41.15 90 top
JP6  30.23,50.8 0 top
L  27.94,42.16 90 top
L1  8.26,45.21 180 top
ON  76.2,36.83 90 top
PC1  18.41,9.14 90 top
PC2  25.53,9.14 90 top
POWER  36.83,2.54 0 top
PWML  54.61,50.8 180 top
R1  40.51,14.61 90 top
R2  18.41,29.34 0 top
RESET  74.17,27.94 90 top
RESET-EN  27.94,15.75 0 top
RN1  80.64,36.83 270 top
RN2  12.06,37.08 90 top
RN3  27.94,39.37 270 top
RN4  27.94,31.11 90 top
RN5  18.41,16.51 90 top
RX  27.94,34.29 90 top
T1  9.14,25.91 270 top
TX  27.94,36.58 90 top
U$1  not placed on the board
X1  5.33,8.38 90 top
X2  3.81,38.1 270 top
XIO  95.25,29.21 270 top
Y1  38.35,14.61 270 top
Y2  18.41,26.04 180 top
Z1  12.06,34.29 0 top
Z2  12.06,39.88 0 top

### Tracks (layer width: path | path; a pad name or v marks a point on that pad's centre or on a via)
8PB4
  Top 0.254: 20.57,39.88 JP5.1 21.19,39.52 IC4.18
8PB5
  Top 0.254: 19.56,41.15 19.56,39.42 20.69,38.29 IC4.19
  Top 0.305: 19.56,41.15 JP5.3
8PB6
  Top 0.254: IC4.20 20.19,38.1 18.41,39.88 JP5.2
8PB7
  Top 0.254: IC4.21 19.68,37.85 19.05,38.48 17.78,38.48 17.02,39.24 17.02,39.37
  Top 0.305: 17.02,39.37 17.02,41.15 JP5.4
+3V3  (via drill 0.41)
  Top 0.305: IC7.6 15.42,21.66 15.11,21.97 15.11,22.86 15.75,23.5 23.11,23.5 v24.64,21.97
  Top 0.406: 28.89,21.62 IC6.5
  Top 0.61: POWER.4 35.56,9.27 v34.67,10.16 | 28.89,21.62 C13.2 28.96,21.55 28.96,20.95 28.45,20.45 25.15,20.45 24.64,20.95 v24.64,21.97
  Bottom 0.61: v34.67,10.16 34.29,10.16 33.91,10.54 31.11,10.54 27.94,13.72 22.48,13.72 20.95,15.24 20.95,18.29 24.26,21.59 24.26,21.72 v24.64,21.97
+5V  (via drill 0.41)
  Top 0.254: IC3.80 54.81,36.3 54.79,36.27 54.81,36.25 54.81,35.41 | 57.66,27.3 57.7,27.35 | v28.07,28.07 28,28.19 27.94,28.64 27.94,31.37 27.79,31.52 RN4.6 RN4.5 | RN5.8 18.23,15.31 18.41,15.49 18.41,16 18.52,16.11 RN5.2 | IC4.32 16.41,33.05 16,32.64
  Top 0.305: 54.86,34.67 54.86,35.1 54.81,35.15 54.81,35.41 | 57.7,27.35 IC3.61 | v57.02,26.67 57.66,27.3 | 44.45,30.48 43.94,29.85 IC3.10 41.59,29.85 C6.1 | IC3.100 44.17,36.35 v43.69,36.7 | 83.31,36.45 82.17,36.45 | v24.64,40.13 26.42,40.13 26.74,40.51 RN3.1 | RN1.6 82.15,36.43 82.17,36.45 | 82.17,36.45 82.17,37.21 82.15,37.23 RN1.7 | C9.1 13.97,30.35 v15.24,30.35 | RN5.2 23.6,16.11 v23.88,16.38 | IC4.4 19.69,31.62 20.07,31.24 v22.61,31.24 | D2.C 14.15,44.53 14.99,43.69 19.56,43.69 ICSP1.2 | D3.C 34.49,12.9 34.29,12.7 32.64,12.7 32.43,12.9 31.93,12.9 31.62,13.21
  Top 0.406: 44.55,30.7 44.45,30.48 v44.58,30.86 | 47.3,22.41 IC3.31 | C5.1 58.04,35.97 56.52,34.42 56.49,34.39 v56.49,34.16 | C11.2 25.53,29.09 26.99,27.62 | C11.2 25.65,29.59 24.13,31.11 22.73,31.11 v22.61,31.24 | C11.2 24.51,28.19 23.96,28.19 22.86,26.96 22.86,24.26 22.61,24.13 15.37,24.13 14.48,23.24 14.48,21.34 15.37,20.45 16.22,20.45 IC7.8 | 16,32.64 16,31.11 v15.24,30.35
  Top 0.508: 47.3,22.41 47.5,22.61 52.96,22.61 v57.02,26.67 | 26.96,26.67 IC6.3 26.99,27.62 27.3,27.94 27.94,27.94 | IC6.1 28.89,27.24 v28.07,28.07
  Top 0.61: v28.07,28.07 27.94,27.94 | 54.86,34.67 54.86,34.29 54.99,34.16
  Top 0.813: 9.27,17.78 IC1.2 | C4.1 37.72,3.94 POWER.5 | 83.31,34.8 83.31,34.92 | 65.41,32.26 65.41,31.24 ICSP.2 | T1.2 10.11,26.85 8.89,27.94
  Top 1.27: XIO.1 XIO.2 | v63.14,34.14 63.37,33.53 64.64,32.26 65.41,32.26 67.31,32.26 69.09,34.04 82.55,34.04 83.31,34.8 | 83.31,34.92 83.31,36.45 83.44,36.7 v83.44,39.12 | 44.55,30.7 44.55,31.34 45.09,31.75 52.32,31.75 54.74,34.16 54.99,34.16 v56.49,34.16 | v31.62,14.61 31.62,13.21 31.62,12.57 28.13,9.08 | v29.21,4.95 29.21,6.48 28.83,6.48 28.32,6.99 28.32,8.51 28.13,9.08 | PC2.+ 25.53,10.92 26.54,9.91 27.05,9.65 28.13,9.08
  Bottom 0.406: v44.58,30.86 44.58,30.73 43.69,31.62 v43.69,36.7 | 61.47,30.1 60.07,30.1 57.02,27.05 v57.02,26.67 | 23.5,41.15 16.76,41.15 16.64,41.27 16.26,41.27 | 17.27,43.69 20.19,43.69 | v23.88,16.38 30.1,16.38 | POWER.2 30.48,3.68 v29.21,4.95
  Bottom 0.61: 63.12,34.16 v63.14,34.14 | 23.62,41.27 23.5,41.15 | 16.26,41.27 16.89,41.78 16.89,43.31 17.27,43.69 | 20.19,43.69 20.83,44.32 ICSP1.2 | v15.24,30.35 16.13,31.24 v22.61,31.24 22.61,32.89 17.78,37.72 17.27,37.72 16.38,38.61 15.88,38.61 15.11,39.37 15.11,41.27
  Bottom 0.813: 61.47,30.1 62.1,30.73 62.1,33.27 v63.14,34.14
  Bottom 1.016: 91.19,48.01 91.69,48.26 92.84,49.4 92.96,49.78
  Bottom 1.27: v29.21,4.95 36.2,4.95 37.47,3.68 POWER.5 | v56.49,34.16 63.12,34.16 | v44.58,30.86 43.56,30.86 42.93,30.23 42.93,28.83 41.53,27.43 37.47,27.43 32.77,22.73 30.1,22.73 | ICSP1.2 20.95,44.83 21.59,44.45 22.86,43.18 22.86,42.04 23.62,41.27 23.62,41.15 v24.64,40.13 27.18,37.59 27.18,28.96 v28.07,28.07 28.96,27.18 29.97,26.29 29.97,22.73 30.1,22.73 | 30.1,22.73 30.1,16.38 30.1,16 v31.62,14.61 | v83.44,39.12 87.38,43.05 87.38,44.32 91.06,48.01 91.19,48.01 | v8.89,29.21 8.26,29.84 8.26,31.75 4.45,35.56 4.45,40.39 5.33,41.27 15.11,41.27 16.26,41.27 | 92.96,49.78 XIO.1
  other vias: 6.35,22.23 4.45,22.23 8.26,22.23 2.54,22.23 8.89,19.68 2.54,13.97 6.35,13.97 4.45,13.97 8.89,15.88 8.26,13.97
  pour Top (isolate 0.406, no thermals): 9.53,13.34 9.53,29.84 0.64,29.84 0.64,13.34
  pour Bottom: 1.27,13.34 1.27,29.84 10.79,29.84 10.79,13.34
ADC0  (via drill 0.41)
  Top 0.203: IC3.97 46.3,37.52 45.47,38.35 v45.47,38.86
  Bottom 0.203: ADCL.1 50.8,3.3 52.7,5.21 52.7,9.4 49.15,12.95 49.15,22.35 46.23,25.27 46.23,37.59 45.47,38.35 v45.47,38.86
ADC1  (via drill 0.41)
  Top 0.203: IC3.96 46.8,37.66 46.48,37.97 46.48,39.24 46.1,39.62 v46.1,40.01
  Bottom 0.203: ADCL.2 53.34,9.6 49.63,13.31 49.63,22.55 46.74,25.45 46.74,37.72 46.48,37.97 46.48,39.24 46.1,39.62 v46.1,40.01
ADC2  (via drill 0.41)
  Top 0.203: v46.99,40.89 46.99,38.1 47.27,37.82 47.27,36.68 47.37,36.58 47.3,36.51 47.3,36.38 47.27,36.35 | 47.27,36.35 47.24,36.32 | 47.27,36.35 IC3.95
  Bottom 0.203: ADCL.3 55.88,7.8 50.22,13.46 50.22,22.68 47.27,25.63 47.27,37.82 46.99,38.1 v46.99,40.89
ADC3  (via drill 0.41)
  Top 0.203: IC3.94 47.8,37.92 47.5,38.23 47.5,40.13 47.88,40.51 v47.88,41.78
  Bottom 0.203: ADCL.4 58.42,2.74 58.52,2.85 58.52,3.05 58.42,3.15 58.42,6.02 50.75,13.69 50.75,22.86 47.8,25.81 47.8,37.85 47.75,37.97 47.5,38.23 47.5,40.13 47.88,40.51 v47.88,41.78
ADC4  (via drill 0.41)
  Top 0.203: IC3.93 48.3,38.06 48.01,38.35 48.01,40.01 48.39,40.39 48.39,41.15 48.77,41.53 v48.77,42.67
  Bottom 0.203: 60.96,2.44 ADCL.5 60.96,4.27 51.26,13.97 51.26,23.06 48.31,26.01 48.31,38.05 48.01,38.35 48.01,40.01 48.39,40.39 48.39,41.15 48.77,41.53 v48.77,42.67
ADC5  (via drill 0.41)
  Top 0.203: IC3.92 48.8,38.2 48.51,38.48 48.51,39.75 48.9,40.13 48.9,41.02 49.28,41.4 49.28,42.04 49.66,42.42 v49.66,43.56
  Bottom 0.203: v49.66,43.56 49.66,42.42 49.28,42.04 49.28,41.4 48.9,41.02 48.9,40.13 48.51,39.75 48.51,38.48 48.77,38.23 48.77,26.16 51.82,23.11 51.82,14.22 61.47,4.57 62.1,4.57 63.5,3.17 ADCL.6
ADC6  (via drill 0.41)
  Top 0.203: IC3.91 49.3,39.35 v49.28,39.37
  Bottom 0.203: v49.28,39.37 49.28,26.29 52.32,23.24 52.32,14.48 61.47,5.21 62.23,5.21 62.99,4.45 64.14,4.45 ADCL.7
ADC7  (via drill 0.41)
  Top 0.203: IC3.90 49.8,38.62 50.16,38.99 50.16,39.62 49.66,40.13 49.66,41.15 50.42,41.91 v50.42,42.29
  Bottom 0.203: v50.42,42.29 50.42,41.91 49.66,41.15 49.66,40.13 50.16,39.62 50.16,38.99 49.78,38.61 49.78,26.42 52.83,23.37 52.83,14.61 61.47,5.97 62.23,5.97 63.12,5.08 64.14,5.08 64.77,4.45 67.31,4.45 68.58,3.17 | 68.58,3.17 ADCL.8 | 68.58,3.17 68.58,3.94
ADC8  (via drill 0.41)
  Top 0.203: IC3.89 50.3,38.49 50.67,38.86 50.67,40.26 v50.42,40.51
  Bottom 0.203: v50.42,40.51 50.67,40.26 50.67,38.86 50.29,38.48 50.29,26.54 53.34,23.5 53.34,14.86 61.72,6.48 62.48,6.48 63.25,5.71 64.14,5.71 64.9,4.95 69.98,4.95 71.75,3.17 73.66,3.17 ADCH.1
ADC9  (via drill 0.41)
  Top 0.203: IC3.88 50.8,38.35 51.18,38.73 51.18,42.55 51.31,42.67 v51.31,43.18
  Bottom 0.203: v51.31,43.18 51.31,42.67 51.18,42.55 51.18,38.73 50.8,38.35 50.8,26.67 53.85,23.62 53.85,15.11 57.91,11.05 66.55,11.05 73.03,4.57 75.44,4.57 76.2,3.81 ADCH.2
ADC10  (via drill 0.41)
  Top 0.203: IC3.87 51.3,38.22 51.69,38.61 51.69,41.15 51.94,41.4 v51.94,42.04
  Bottom 0.203: v51.94,42.04 51.94,41.4 51.69,41.15 51.69,38.61 51.31,38.23 51.31,26.8 54.36,23.75 54.36,15.37 58.04,11.68 66.67,11.68 73.15,5.21 77.85,5.21 78.74,4.32 ADCH.3
ADC11  (via drill 0.41)
  Top 0.203: IC3.86 51.8,38.08 52.2,38.48 52.2,41.02 52.7,41.53 52.7,42.42 52.32,42.8 v52.32,44.07
  Bottom 0.203: v52.32,44.07 52.32,42.8 52.7,42.42 52.7,41.53 52.2,41.02 52.2,38.48 51.82,38.1 51.82,26.92 54.86,23.88 54.86,15.62 58.17,12.32 66.8,12.32 73.28,5.84 79.5,5.84 81.28,4.06 ADCH.4
ADC12  (via drill 0.41)
  Top 0.203: IC3.85 52.3,37.95 52.7,38.35 52.7,40.89 53.21,41.4 v53.21,43.18
  Bottom 0.203: v53.21,43.18 53.21,41.4 52.7,40.89 52.7,38.35 52.32,37.97 52.32,27.05 55.37,24 55.37,15.88 58.29,12.95 66.93,12.95 73.53,6.35 79.88,6.35 81.79,4.45 83.44,4.45 83.82,4.06 ADCH.5
ADC13  (via drill 0.41)
  Top 0.203: IC3.84 52.8,37.81 53.21,38.23 53.21,40.77 53.72,41.27 53.72,42.42 54.1,42.8 v54.1,44.2
  Bottom 0.203: v54.1,44.2 54.1,42.8 53.72,42.42 53.72,41.27 53.21,40.77 53.21,38.23 52.83,37.85 52.83,27.18 55.88,24.13 55.88,16.13 58.42,13.59 67.18,13.59 73.91,6.86 80.26,6.86 82.04,5.08 85.22,5.08 86.36,3.94 ADCH.6
ADC14  (via drill 0.41)
  Top 0.203: IC3.83 53.3,37.68 53.72,38.1 53.72,40.51 54.61,41.4 v54.61,42.04
  Bottom 0.203: v54.61,42.04 54.61,41.4 53.72,40.51 53.72,38.1 53.34,37.72 53.34,27.3 56.39,24.26 56.39,16.38 58.55,14.22 67.44,14.22 74.3,7.37 80.64,7.37 82.3,5.71 87.25,5.71 88.9,4.06 ADCH.7
ADC15  (via drill 0.41)
  Top 0.203: IC3.82 53.8,37.54 54.23,37.97 54.23,39.88 v54.61,40.26
  Bottom 0.203: v54.61,40.26 54.23,39.88 54.23,37.97 53.85,37.59 53.85,27.43 56.9,24.38 56.9,16.64 58.67,14.86 67.69,14.86 74.68,7.87 81.03,7.87 82.55,6.35 89.03,6.35 91.44,3.94 ADCH.8
AREF  (via drill 0.41)
  Top 0.203: C3.1 25.53,44.45 24.77,45.21 24.77,49.15 23.88,50.04 JP6.3
  Top 0.254: IC3.98 45.8,37.38 45.34,37.85 45.09,37.85 44.32,38.48 v42.34,38.48
  Top 0.305: v28.19,45.85 27.73,45.59 C3.1
  Bottom 0.305: v28.19,45.85 28.83,45.34 41.91,45.34 42.55,44.7 42.55,38.66 v42.34,38.48
CMP
  Top 0.203: C12.2 20.7,17.4 18.03,20.07 18.03,21.84 17.57,22.31 IC7.5
  Top 0.254: 19.07,16.89 18.54,16.89 18.41,17.02 18.41,17.53 18.23,17.71 RN5.5
  Top 0.305: 19.07,16.89 RN5.3 | RN5.3 19.87,16.91 | C12.2 20.47,16.91 RN5.3
D+
  Top 0.406: 6.99,40.64 7.2,40.85 9.06,40.85 10.03,39.88 10.03,38.73 10.41,38.35 11.32,38.35 RN2.5 11.61,38.28 12.06,38.73 12.06,39.12 12.45,39.5 12.94,39.5 Z2.2
  Top 0.61: X2.3 6.52,40.17 6.99,40.64
D-
  Top 0.406: 9.53,38.1 9.56,38.1 10.03,37.63 10.03,37.59 10.79,35.81 11.32,35.81 RN2.8 12.73,34.54 Z1.2
  Top 0.61: X2.2 8.53,39.1 9.53,38.1
DTR  (via drill 0.41)
  Top 0.254: 24.26,38.17 23.81,38.17 v23.75,38.23 | 24.26,38.17 RN3.4 | IC4.13 24.25,35.05 25.02,35.81 25.02,37.41 24.26,38.17
  Top 0.305: C7.1 26.04,18.29 v25.78,18.16
  Bottom 0.254: v25.78,18.16 25.91,18.16 27.18,19.43 27.18,25.4 25.02,27.56 25.02,36.96 v23.75,38.23
GATE_CMD
  Top 0.305: T1.3 10.29,24.79 10.29,21.72 10.79,21.21 12.95,21.21 13.21,20.95 13.84,20.95 15.49,19.3 17.02,19.3 17.53,19.81 17.53,20.7 17.22,21.01 IC7.7
  Top 0.406: T1.3 10.16,24.64
GND  (via drill 0.41)
  Top 0.203: 54.23,35.18 54.3,35.25 IC3.81 54.33,36.35 | 54.3,37.28 54.3,36.38 54.33,36.35 | IC3.32 47.8,21.39 47.88,21.46 52.83,21.46 | IC3.32 | IC3.32 47.8,19.48 46.99,18.67 | 54.33,36.35 54.36,36.32
  Top 0.305: IC1.1 11.81,15.49 | 45.39,35.1 45.29,35.2 IC3.99 | IC3.11 42.86,29.35 42.88,29.36 44.32,29.36 | 44.32,29.36 44.4,29.36 | 56.06,27.86 56.08,27.84 58.81,27.84 | 58.83,27.84 58.82,27.85 IC3.62 58.81,27.84 | 54.3,37.28 55.24,38.23 v55.24,38.86 | 44.32,29.36 44.32,29.34 44.35,29.36 44.42,29.36 | v38.35,29.23 38.61,30.48 | 59.94,27.81 59.92,27.84 58.81,27.84 | v18.82,33.68 19.23,33.68 | C15.2 22.48,29.46 21.46,30.48 19.94,30.48 19.19,31.23 IC4.3 | IC4.33 19.94,33.33 v18.82,33.68 | v18.82,33.68 19.19,33.31 | 19.19,32.33 19.19,33.33 v18.82,33.68 | RN5.4 19.09,17.99 18.54,18.54 18.16,18.54 v17.91,18.8
  Top 0.406: C4.2 39.88,6.48 40.26,6.1 40.26,3.94 POWER.6 | 56.06,27.86 56.01,27.81 v55.88,27.94 | v45.21,33.4 45.21,34.92 45.39,35.1
  Top 0.61: v55.88,27.94 55.88,27.81 | 44.42,29.36 v45.09,28.7
  Top 0.813: XIO.35 XIO.36
  Bottom 0.305: GROUND.2 10.16,33.02
  Bottom 0.406: v45.09,28.7 45.09,29.08 | v55.24,38.86 55.24,37.97 54.48,37.21 | v55.88,27.94 54.48,29.34
  Bottom 0.813: v60.83,31.37 59.87,31.37 58.98,30.48 58.93,30.48 56.39,27.94 v55.88,27.94 | 93.73,7.87 XIO.35
  Bottom 1.016: POWER.7 43.18,5.08
  other vias: 69,20 38.23,21.21 32.38,33.66 87.63,38.61 90.17,21.59 72.49,35.71 23.62,11.68 13.59,13.97 32.26,16.38 40.77,21.21 17.02,46.23 25.53,24.26 58.29,41.4 77.5,47.8 44.83,40.13 44.7,27.3 48.39,5.67 25.78,3.43 13.21,22.1 24.13,26.54 25.15,43.31 60.83,27.81 58.04,20.45 12.06,28.19 37.72,24.64 77.98,27.69 76.71,18.04 99.81,31.75 79.88,23.88 69.85,23.5 72.52,27.18 18.41,26.04 69.71,32.1 63,20 99.81,16.51 66.04,50.8 43.67,50.8 13.97,32.26 64.36,38.89 68.71,26.54 37.34,17.02 31.88,20.83 22.35,22.23 45.97,10.49
  pour Top (isolate 0.305, rank 2): 0.64,52.7 101.6,52.7 101.6,0.64 0.64,0.64 0.64,29.84 10.79,29.84 10.79,46.35 0.64,46.35
  pour Bottom (isolate 0.305, rank 2): 0.64,52.7 101.6,52.7 102.23,52.07 102.23,0.64 1.27,0.64 0.64,1.27 0.64,29.84 10.79,29.84 10.79,46.35 0.64,46.35
L13
  Top 0.203: RN3.7 31.01,39.77 31.5,40.26 32.89,40.26 33.27,39.88 33.27,22.99 34.67,21.59 34.67,20.19 34.29,19.81 22.86,19.81 21.97,20.7 | IC7.2 21.79,21.01 21.97,20.83 21.97,20.7 | IC7.1 21.8,20.36 21.97,20.57 21.97,20.7
M8RXD
  Top 0.254: 27.25,30.73 RN4.7 | IC4.9 25.25,33.05 25.4,32.89
  Top 0.305: 27.25,30.73 26.67,30.73 26.29,30.99 26.29,31.88 25.4,32.89
M8TXD
  Top 0.254: 24.83,32.45 24.2,32.45 24.1,32.35 IC4.8
  Top 0.305: 24.83,32.45 25.53,31.75 25.53,30.86 26.42,29.97 27.21,29.97 RN4.8
MISO2
  Top 0.254: IC4.17 21.69,38.96 22.23,39.5 22.23,45.34 20.83,46.74 ICSP1.1
MOSI2  (via drill 0.41)
  Top 0.254: v22.48,46.35 22.86,45.97 22.86,39.37 22.35,38.86 22.35,36.7 22.39,36.61 IC4.16
  Bottom 0.254: ICSP1.4 18.8,44.96 20.07,46.23 22.23,46.23 22.35,46.35 v22.48,46.35
N$1
  pour Top: 0.64,52.7 10.79,52.7 11.18,52.7 11.18,46.86 0.64,46.86
N$2
  Top 0.254: RN3.2 27.76,39.82 27.94,40.01 27.94,41.66 28.19,41.91 L.A
N$3  (via drill 0.41)
  Top 0.203: 77.22,37.08 ON.A | v80.14,46.74 80.01,46.74 79.12,45.85 60.96,45.85 v60.07,46.74
  Top 0.254: v30.48,46.74 30.99,46.23 30.99,42.16 29.34,40.51 28.89,40.51 RN3.8 | 77.22,37.08 77.22,37.37 v75.96,38.62
  Bottom 0.203: v75.96,38.62 80.14,42.8 v80.14,46.74 | v60.07,46.74 59.94,46.74 59.44,46.74 57.66,48.51 51.69,48.51 50.29,47.12 44.7,47.12 43.56,45.97 31.24,45.97 v30.48,46.74
N$54
  Top 0.254: RN4.4 28.61,33.82 RX.A
N$55
  Top 0.254: RN4.3 29.48,31.52 30.23,32.26 30.23,35.18 28.99,36.41 TX.A
PA0
  Top 0.203: IC3.78 55.8,37.89 56.26,38.35 56.26,43.18 58.42,45.34 90.3,45.34 93.22,48.26 XIO.3
PA1
  Top 0.203: IC3.77 56.3,37.63 56.77,38.1 56.77,42.93 58.67,44.83 90.81,44.83 92.96,46.99 95.25,46.99 XIO.4
PA2
  Top 0.203: XIO.5 92.71,45.72 91.31,44.32 58.93,44.32 57.28,42.67 57.28,37.85 56.8,37.37 IC3.76
PA3
  Top 0.203: XIO.6 95.25,44.45 92.2,44.45 91.57,43.81 61.98,43.81 61.34,43.18 61.34,39.26 59.44,37.35 59.44,34.67 59.11,34.35 IC3.75
PA4
  Top 0.203: IC3.74 59.75,33.85 59.94,34.04 59.94,37.23 61.85,39.13 61.85,42.8 62.36,43.31 92.58,43.31 92.71,43.18 XIO.7
PA5
  Top 0.203: IC3.73 60.02,33.35 60.45,33.78 60.45,36.97 62.36,38.88 62.36,42.29 62.87,42.8 91.57,42.8 92.46,41.91 95.25,41.91 XIO.8
PA6
  Top 0.203: IC3.72 60.28,32.85 60.96,33.53 60.96,36.72 62.87,38.62 62.87,41.91 63.25,42.29 90.81,42.29 92.46,40.64 XIO.9
PA7
  Top 0.203: IC3.71 60.54,32.35 61.47,33.27 61.47,36.47 63.37,38.37 63.37,41.4 63.75,41.78 90.04,41.78 92.46,39.37 95.25,39.37 XIO.10
PB0  (via drill 0.41)
  Top 0.203: IC3.19 45.39,25.35 v45.21,25.4 | v49.4,11.56 49.53,11.56 49.78,11.81 92.33,11.81 92.71,11.43 95.25,11.43 XIO.34
  Bottom 0.203: v45.21,25.4 45.34,25.4 48.64,22.1 48.64,12.19 v49.4,11.56
PB1  (via drill 0.41)
  Top 0.203: IC3.20 41.19,24.85 v40.89,25.15 | XIO.33 92.71,10.16 91.57,11.3 75.18,11.3 74.8,10.92 v73.91,10.92 73.53,11.3 50.55,11.3 49.53,10.29 v49.23,10.29
  Bottom 0.203: v40.89,25.15 44.2,25.15 45.97,23.37 46.61,23.37 48.13,21.84 48.13,10.92 48.77,10.29 v49.23,10.29 | 63.75,27.94 64.69,27 64.69,18.31 67,16
  Bottom 0.254: 63.75,27.94 ICSP.3
  Bottom 0.305: 67,16 68.83,16 v73.91,10.92
PB2  (via drill 0.41)
  Top 0.203: IC3.21 41.24,24.35 41.02,24.13 v39.88,24.13 | XIO.32 97.79,11.43 97.79,9.53 97.16,8.89 92.71,8.89 90.81,10.79 77.47,10.79 76.83,10.16 v75.82,10.16 75.69,10.03 73.66,10.03 72.9,10.79 51.34,10.79 v50.67,10.12
  Bottom 0.203: v39.88,24.13 41.02,24.13 41.66,24.64 44.07,24.64 45.85,22.86 46.35,22.86 47.62,21.59 47.62,10.54 48.77,9.4 49.95,9.4 v50.67,10.12 | ICSP.4 66.42,27.94 67.31,27.05
  Bottom 0.254: 67.31,27.05 67.31,24.77 65.66,23.11 65.66,19.11 67.49,17.27
  Bottom 0.305: 67.49,17.27 69.85,17.27 75.82,11.3 v75.82,10.16
PB3  (via drill 0.41)
  Top 0.203: IC3.22 44.35,23.85 44.58,23.62 v44.58,22.99 | v81.03,8.76 81.03,9.14 80.01,10.16 77.85,10.16 77.09,9.4 73.53,9.4 72.59,10.34 52.12,10.34 50.42,8.64 v49.02,8.64
  Bottom 0.203: v81.03,8.76 81.15,8.76 82.93,6.99 89.66,6.99 91.19,5.46 96.9,5.46 98.04,6.6 98.04,10.54 97.16,11.43 95.25,11.43 XIO.31 | v44.58,22.99 45.09,22.99 45.72,22.35 46.1,22.35 47.12,21.34 47.12,10.29 48.77,8.64 v49.02,8.64 | ICSP.1 64.97,29.13 64.97,27.38 65.1,27.25 65.1,18.72 67.18,16.64
  Bottom 0.254: v81.03,8.76 81.03,9.27 80.52,9.78 77.98,9.78 77.34,9.14 75.56,9.14 74.93,9.78 74.93,11.18 74.17,11.94 | 69.47,16.64 67.18,16.64
  Bottom 0.305: 74.17,11.94 69.47,16.64
PB4
  Top 0.203: IC3.23 42.9,23.35 42.93,23.37 36.32,23.37 35.31,24.38 35.31,47.62 36.58,48.9 JP6.8
PB5
  Top 0.203: IC3.24 36.08,22.85 34.8,24.13 34.8,48.51 34.04,49.28 JP6.7
PB6
  Top 0.203: IC3.25 42.92,22.35 42.93,22.35 35.81,22.35 34.29,23.88 34.29,47.62 31.75,50.16 JP6.6
PB7  (via drill 0.41)
  Top 0.203: 35.15,20.22 37.59,20.22 | 37.59,20.22 44.09,20.22 44.22,20.34 IC3.26 | v30.86,40.77 33.15,40.77 33.78,40.13 33.78,23.24 35.15,21.87 35.15,20.22 | 37.59,20.22 37.57,20.19 | IC7.3 20.46,21.59 19.81,21.59 19.43,21.21 19.43,20.19 20.32,19.3 34.42,19.3 35.15,20.04 35.15,20.22
  Bottom 0.254: JP6.5 29.21,49.53 26.67,46.99 26.67,45.09 28.57,43.18 28.57,43.05 v30.86,40.77
PC0
  Top 0.203: IC3.53 61.49,23.35 62.74,22.1 81.03,22.1 88.14,29.21 95.25,29.21 XIO.18
PC1
  Top 0.203: IC3.54 61.75,23.85 62.87,22.61 80.52,22.61 88.39,30.48 XIO.17
PC2
  Top 0.203: IC3.55 62.01,24.35 63.25,23.11 68.07,23.11 69.98,25.02 82.04,25.02 88.77,31.75 95.25,31.75 XIO.16
PC3
  Top 0.203: IC3.56 62.28,24.85 63.5,23.62 67.82,23.62 69.72,25.53 81.53,25.53 89.03,33.02 XIO.15
PC4
  Top 0.203: IC3.57 61.85,25.35 62.99,26.48 67.39,26.48 69.98,29.08 83.82,29.08 89.03,34.29 95.25,34.29 XIO.14
PC5
  Top 0.203: IC3.58 61.66,25.85 62.66,26.86 66.98,26.86 69.85,29.72 83.57,29.72 89.41,35.56 XIO.13
PC6
  Top 0.203: IC3.59 61.52,26.35 62.48,27.3 62.48,28.7 62.79,29.02 68.28,29.02 69.62,30.35 83.19,30.35 89.66,36.83 95.25,36.83 XIO.12
PC7
  Top 0.203: IC3.60 61.39,26.85 61.98,27.43 61.98,28.83 62.56,29.4 67.87,29.4 69.32,30.86 82.68,30.86 89.92,38.1 XIO.11
PD7
  Top 0.203: XIO.19 88.01,27.94 81.66,21.59 60.3,21.59 60.3,21.57 59.69,20.95 59.69,20.57 58.17,19.05 58.04,19.05 57.4,18.41 56.9,18.41 56.8,18.51 IC3.50
PE0  (via drill 0.41)
  Top 0.203: PWML.1 61.47,48.77 58.42,48.77 56.77,47.12 51.31,47.12 49.66,45.47 45.85,45.47 45.72,45.34 40.77,45.34 40.39,44.96 40.39,36.7 v40.64,36.45 42.16,34.92 43.56,34.92 43.94,34.54 43.94,34.04 43.75,33.85 IC3.2
  Top 0.254: v30.61,37.47 30.54,37.4 30.54,35.74 30.86,35.43 30.86,31.88 29.72,30.73 28.63,30.73 RN4.2
  Bottom 0.254: v30.61,37.47 39.62,37.47 v40.64,36.45
PE1  (via drill 0.41)
  Top 0.203: v40.39,35.18 39.88,35.69 39.88,45.09 40.64,45.85 45.34,45.85 45.47,45.97 49.28,45.97 50.93,47.62 56.52,47.62 58.17,49.28 59.69,49.28 60.96,50.55 PWML.2 | v39.62,33.53 39.88,33.27 39.95,33.35 IC3.3
  Top 0.254: RN4.1 29.91,29.91 31.5,31.5 v31.5,36.32
  Bottom 0.203: v40.39,35.18 40.39,34.29 v39.62,33.53
  Bottom 0.254: v31.5,36.32 39.24,36.32 v40.39,35.18
PE3  (via drill 0.41)
  Top 0.203: IC3.5 39.54,32.35 38.86,33.02 38.86,45.34 40.39,46.86 44.7,46.86 45.09,47.24 46.61,47.24 v47.24,48.01
  Bottom 0.203: PWML.6 50.67,50.8 47.88,48.01 v47.24,48.01
PE4
  Top 0.203: IC3.6 39.02,31.85 38.35,32.51 38.35,45.47 40.26,47.37 44.45,47.37 45.47,48.39 46.48,48.39 46.86,48.77 56.64,48.77 58.42,50.55 PWML.3
PE5
  Top 0.203: IC3.7 42.78,31.35 42.55,31.37 38.73,31.37 37.85,32.26 37.85,45.59 40.13,47.88 44.2,47.88 45.21,48.9 46.35,48.9 46.74,49.28 55.75,49.28 55.88,49.4 PWML.4
PG0  (via drill 0.41)
  Top 0.203: IC3.51 58.8,21.84 v59.05,21.46 | XIO.22 95.25,24.13 88.14,24.13 84.07,20.07 71.75,20.07 71.25,19.56 70.36,18.67 70.1,18.41 59.69,18.41 59.44,18.67 v59.05,18.67
  Bottom 0.203: v59.05,18.67 v59.05,21.46
PG1  (via drill 0.41)
  Top 0.203: IC3.52 60.44,22.85 v60.83,22.48 | XIO.21 88.14,25.4 83.31,20.57 71.12,20.57 69.6,19.05 60.33,19.05 59.94,19.43 v59.94,19.56
  Bottom 0.203: v59.94,19.56 60.58,19.56 61.34,20.32 61.34,21.97 v60.83,22.48
PG2  (via drill 0.41)
  Top 0.203: IC3.70 59.8,31.85 59.92,31.73 59.92,29.49 v60.33,29.08 | v60.58,20.7 61.09,20.7 61.47,21.08 82.55,21.08 88.14,26.67 95.25,26.67 XIO.20
  Bottom 0.203: v60.58,20.7 60.2,20.7 59.94,20.95 59.94,28.57 v60.33,29.08
PG5  (via drill 0.41)
  Top 0.203: IC3.1 42.73,34.35 42.67,34.29 40.13,34.29 39.37,35.05 39.37,45.21 40.51,46.35 44.96,46.35 45.09,46.48 48.26,46.48 v49.66,47.88
  Bottom 0.203: PWML.5 53.21,50.8 50.29,47.88 v49.66,47.88
PH3
  Top 0.203: IC3.15 37.42,27.35 37.34,27.43 37.34,45.72 40.01,48.39 43.94,48.39 44.96,49.35 46.23,49.35 47.62,50.8 PWML.7
PH4
  Top 0.203: IC3.16 37.16,26.85 36.83,27.18 36.83,45.85 39.88,48.9 43.69,48.9 45.59,50.8 PWML.8
PH5
  Top 0.203: IC3.17 36.9,26.35 36.32,26.92 36.32,46.1 39.62,49.4 41.15,49.4 41.66,49.91 JP6.10
PH6
  Top 0.203: IC3.18 42.73,25.85 42.67,25.91 36.58,25.91 35.81,26.67 35.81,46.86 39.12,50.16 JP6.9
PL0
  Top 0.203: 49.28,20.3 49.28,14.22 51.18,12.32 90.3,12.32 91.95,13.97 95.25,13.97 XIO.30
  Top 0.254: IC3.35 49.3,20.32 49.28,20.3
PL1
  Top 0.203: IC3.36 49.8,14.46 51.44,12.83 89.53,12.83 91.95,15.24 XIO.29
PL2
  Top 0.203: 50.29,20.3 50.29,14.99 51.94,13.34 88.9,13.34 92.08,16.51 95.25,16.51 XIO.28
  Top 0.254: IC3.37 50.27,20.32 50.29,20.3
PL3
  Top 0.203: IC3.38 50.8,15.49 52.45,13.84 88.27,13.84 92.2,17.78 XIO.27
PL4
  Top 0.203: 51.31,20.22 51.31,15.75 52.7,14.35 87.63,14.35 92.33,19.05 95.25,19.05 XIO.26
  Top 0.254: IC3.39 51.3,20.28 51.33,20.24 51.31,20.22
PL5
  Top 0.203: IC3.40 51.8,16.02 52.96,14.86 87,14.86 92.46,20.32 XIO.25
PL6
  Top 0.203: 52.32,20.24 52.32,16.51 53.47,15.37 86.49,15.37 92.71,21.59 95.25,21.59 XIO.24
  Top 0.254: IC3.41 52.3,20.32 52.27,20.3 52.32,20.24
PL7
  Top 0.203: IC3.42 52.8,17.05 53.98,15.88 85.72,15.88 92.71,22.86 XIO.23
PWRIN
  Top 1.016: D1.A 18.29,2.79 17.02,4.06 17.02,4.19 15.37,5.84 15.24,5.84 13.46,7.62 12.37,7.62 X1.2
RD+
  Top 0.254: RN2.4 13.4,38.28 13.59,38.1 13.59,37.97 14.48,37.08 14.48,36.07 16,34.55 IC4.29
RD-
  Top 0.254: RN2.1 13.28,35.85 13.5,35.85 13.97,35.38 13.97,35.05 14.97,34.05 IC4.30
RESET  (via drill 0.41)  (1 unrouted)
  Top 0.254: 46.8,19.44 46.53,19.18 44.2,19.18 43.69,19.68 | 64.85,24.18 67.61,24.18 69.47,26.04 78.74,26.04 v80.01,27.3 | 28.79,17.87 28.16,17.87 27.3,17.02 27.3,15.88 RESET-EN.1
  Top 0.305: POWER.3 33.02,7.87 v31.5,9.4 | 46.8,19.44 IC3.30 | ICSP.5 64.85,24.18 | 43.69,19.68 36.2,19.68 35.56,19.05 35.56,18.8 | RESET.4 v80.01,32.13 | 28.79,17.87 C7.2 | RESET-EN.1 RESET-EN.2 | RESET-EN.1 27.3,15.37 | 35.56,18.8 D3.A 34.34,16.3 C1.1 | RESET-EN.2 28.7,16.64 30.86,18.8 35.56,18.8 | RN5.1 26.74,15.31 RESET-EN.1 | RESET-EN.2 28.7,12.83 v28.07,12.19
  Top 0.406: v46.85,8.26 47.88,8.26 48.51,7.62 49.53,7.62 49.91,8 50.55,8 52.43,9.83 72.08,9.83 73.28,8.64 78.49,8.64 v78.61,8.76
  Bottom 0.254: 63.75,25.27 64.26,24.77 64.26,17.78 66.67,15.37
  Bottom 0.305: v78.61,8.76 78.11,8.76 77.98,8.64 74.93,8.64 68.2,15.37 66.67,15.37 | 63.75,25.27 ICSP.5 | v46.85,8.26 45.72,9.27 31.62,9.27 v31.5,9.4 30.86,9.4 v28.07,12.19 | v80.01,27.3 v80.01,32.13
RESET2  (via drill 0.41)
  Top 0.254: IC4.24 16.51,38.93 16.51,39.12 | RN5.7 17.38,16.11 v16.51,15.24
  Top 0.305: ICSP1.5 14.99,47.5 | v16.51,15.24 16.58,15.31 | 16.51,39.12 16.51,39.5 v16.19,39.81 16.26,39.75 16.26,41.4 14.35,43.31 12.19,43.31 11.56,43.94 11.56,46.4 D2.A
  Top 0.61: D2.A 13.64,47.5 ICSP1.5
  Bottom 0.305: v16.51,15.24 16.76,15.24 16.76,21.21 19.43,23.75 19.43,29.08 20.57,30.23 23.24,30.23 23.5,30.48 23.5,33.13 18.15,38.48 17.65,38.48 16.45,39.69 v16.19,39.81
RXD1  (via drill 0.41)
  Top 0.203: IC3.45 54.33,20.35 54.36,20.32 54.36,18.29 55.3,17.35 71.96,17.35 v72.64,17.91
  Bottom 0.203: COMMUNICATION.3 81.28,42.67 74.17,35.56 74.17,19.56 v72.64,17.91
RXD2  (via drill 0.41)
  Top 0.203: IC3.12 41.04,28.85 v41.02,28.83
  Bottom 0.203: v41.02,28.83 41.02,29.84 42.93,31.75 42.93,37.34 43.69,38.1 43.69,44.32 45.47,46.1 50.55,46.1 51.94,47.5 56.64,47.5 58.67,45.47 60.71,45.47 63.63,48.39 63.7,48.39 64.59,49.28 67.39,49.28 68.28,48.39 73.66,48.39 74.04,48.77 75.69,48.77 76.2,49.28 COMMUNICATION.5
RXD3  (via drill 0.41)
  Top 0.203: COMMUNICATION.7 71.12,49.53 70.87,49.28 68.33,49.28 66.8,47.75 v66.8,47.37 | v55.75,29.72 55.75,29.46 56.9,28.32 58.8,28.32 IC3.63
  Bottom 0.203: v66.8,47.37 66.8,46.99 55.45,35.51 55.45,33.6 56.13,32.89 56.26,32.89 56.77,32.38 56.77,31.11 56.39,30.73 56.01,30.73 55.63,30.35 55.63,29.84 v55.75,29.72
RXL
  Top 0.254: 26.27,33.67 25.76,33.67 25.63,33.55 IC4.10
  Top 0.305: 26.27,33.67 RX.C
SCK2
  Top 0.254: ICSP1.3 19.43,48.64 22.23,48.64 23.5,47.37 23.5,39.24 22.86,38.61 22.86,37.85 23.5,37.21 23.5,36.45 23.09,36.05 IC4.15
SCL  (via drill 0.41)
  Top 0.203: IC3.43 53.3,17.31 54.23,16.38 74.68,16.38 75.06,16.76 v75.31,16.89 | v41.53,42.67 v45.09,42.67
  Top 0.254: 80.54,37.23 80.64,37.34 80.64,38.86
  Top 0.305: v81.41,39.12 80.9,39.12 80.64,38.86 | 80.54,37.23 RN1.2
  Bottom 0.203: COMMUNICATION.1 86.36,48.9 85.72,48.9 83.82,46.99 83.82,43.18 81.41,40.77 v81.41,39.12 80.01,39.12 75.18,34.29 75.18,17.02 v75.31,16.89 74.68,16.26 72.52,16.26 70.74,18.03 70.74,44.58 67.06,48.26 64.9,48.26 61.09,44.45 57.78,44.45 56.01,46.23 52.2,46.23 51.05,45.09 47.37,45.09 45.34,42.93 v45.09,42.67 | JP6.1 18.8,50.29 19.81,49.28 22.23,49.28 25.65,45.85 25.65,43.94 30.23,39.37 31.5,39.37 32.64,40.51 32.64,42.42 34.42,44.2 40.01,44.2 v41.53,42.67
SDA  (via drill 0.41)
  Top 0.203: v74.04,17.65 73.28,16.89 54.48,16.89 53.85,17.53 53.85,19.94 53.8,20.04 53.8,20.14 IC3.44 | v41.53,44.32 v45.09,44.32
  Top 0.305: v78.74,38.99 78.74,36.83 79.12,36.45 79.95,36.45 RN1.3
  Bottom 0.203: COMMUNICATION.2 83.82,49.53 82.55,48.26 82.55,42.8 v78.74,38.99 74.68,34.92 74.68,18.92 74.04,18.29 v74.04,17.65 74.04,17.02 73.79,16.76 72.64,16.76 71.25,18.16 71.25,44.7 67.18,48.77 64.77,48.77 60.96,44.96 58.29,44.96 56.39,46.86 52.07,46.86 50.8,45.59 46.35,45.59 v45.09,44.32 | JP6.2 21.46,50.8 26.16,46.1 26.16,44.2 30.48,39.88 31.24,39.88 32.13,40.77 32.13,42.67 34.16,44.7 41.15,44.7 v41.53,44.32
TXD1  (via drill 0.41)
  Top 0.203: IC3.46 54.8,20.26 54.86,20.19 54.86,18.67 55.63,17.91 70.74,17.91 v72.01,19.18
  Bottom 0.203: COMMUNICATION.4 78.74,42.55 73.66,37.47 73.66,20.07 72.64,19.18 v72.01,19.18
TXD2  (via drill 0.41)
  Top 0.203: IC3.13 41.81,28.35 41.4,27.94 39.88,27.94 39.75,28.07 v39.75,28.83
  Bottom 0.203: v39.75,28.83 39.75,29.21 42.42,31.88 42.42,37.47 43.18,38.23 43.18,44.7 45.09,46.61 50.42,46.61 51.82,48.01 57.02,48.01 59.05,45.97 60.58,45.97 63.5,48.9 63.63,48.9 64.52,49.78 67.46,49.78 68.35,48.9 73.15,48.9 73.66,49.53 COMMUNICATION.6
TXD3  (via drill 0.41)
  Top 0.203: COMMUNICATION.8 68.33,50.8 67.69,50.16 67.69,49.78 v65.28,47.37 | IC3.64 58.66,28.85 58.55,28.83 57.66,28.83 57.28,29.21 57.28,30.35 v55.75,31.88
  Bottom 0.203: v65.28,47.37 65.28,46.23 54.97,35.89 54.97,32.66 v55.75,31.88
TXL
  Top 0.254: TX.C 26.8,36.83 24.02,34.05 IC4.11
UGND
  Top 0.254: IC4.28 16.39,35.05 15.11,36.32
  Top 0.406: 15.11,36.32 15.11,37.85 14.35,38.61
  Top 0.61: L1.1 10.88,43.69 10.88,42.59 C10.2 11.09,42.12 12.12,41.07 13.89,41.07 14.35,40.51 14.35,38.61
  Top 0.813: X2.4 6.5,36.83 5.08,36.83 4.45,37.47 4.45,40.51 7.75,43.81 8.26,43.81 9.27,44.83 9.27,45.13 L1.1
  Bottom 0.813: X2.4 6.52,36.53 GROUND.1
USBVCC
  Top 0.254: IC4.31 15.89,33.55 15.11,32.77 15.11,32 14.35,31.24
  Top 0.305: 14.35,31.24 13.21,31.24 C8.1
  Top 0.406: C8.1 12.95,31.5 12.32,32.13 10.79,32.13 10.16,31.5 10.16,28.57 11.56,27.18 11.56,25.88
  Top 0.61: 11.56,25.88 T1.1 6.96,24.72 F1.1
USHIELD  (via drill 0.41)
  Top 0.813: X2.P$2 3.81,33.02 5.08,33.02 5.71,33.66 9.79,33.66 Z1.1 | Z2.1 11.06,40.24 9.65,41.66 v9.65,43.18 | L1.2 4.92,45.21 X2.P$1
  Bottom 0.813: v9.65,43.18 4.98,43.18 X2.P$1
  Bottom 1.27: X2.P$2 3.81,33.02 1.91,34.92 1.91,41.27 3.81,43.18 X2.P$1
VIN  (via drill 0.41)
  Top 0.203: 11.77,20.06 IC1.3
  Top 0.305: RN5.6 15.98,16.91 15.75,17.14
  Top 0.813: v24,7.37 22.59,7.37 PC1.+ 17.03,11.54 15.24,13.34 15.24,15.75 15.75,16.26 15.75,17.14 C2.1 12.83,20.06 11.77,20.06
  Top 1.016: D1.C 24,3.01 v24,7.37
  Bottom 1.27: v24,7.37 24.51,7.75 24.89,7.37 44.32,7.37 45.72,5.97 POWER.8
VUCAP
  Top 0.254: 15.11,38.86 15.75,38.23 15.75,36.45 16.65,35.55 IC4.27
  Top 0.305: C10.1 13.17,42.42 14.22,42.42 15.11,41.53 15.11,38.86
XT1
  Top 0.254: 17.8,29.34 R2.1 18.19,30 IC4.1
  Top 0.305: C14.1 16.13,26.29 Y2.2
  Top 0.406: C14.1 R2.1
XT2
  Top 0.254: IC4.2 18.69,29.95 R2.2 | C15.1 20.7,26.29 Y2.1
  Top 0.406: C15.1 R2.2
XTAL1
  Top 0.203: IC3.34 48.8,18.8 47.53,17.53 42.55,17.53
  Top 0.254: Y1.3 39.89,13.61 R1.1 40.89,13.72 41.66,14.48 41.66,16.89 42.29,17.53 42.55,17.53
XTAL2
  Top 0.203: 43.31,18.03 43.41,17.93 47.05,17.93 48.3,19.18 IC3.33
  Top 0.254: 37.83,15.61 Y1.1 37.96,15.61 38.07,15.49 R1.2 41.02,16 41.02,17.14 41.91,18.03 43.31,18.03
XVCC
  Top 0.61: F1.2 2.5,28.62 1.52,29.59 1.52,34.54 1.91,34.92 6.59,34.92 X2.1

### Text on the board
Top: MEGAXL-Rev3b
tPlace: 9 | 8 | 7 | 6 | 5 | 4 | 3 | 2 | 1 | 0 | 22 | 14 | 15 | 16 | 17 | 18 | 19 | 20 | 21 | 13 | 12 | 11 | 10 | 24 | 26 | 28 | 30 | 31 | 32 | 33 | 34 | 35 | 36 | 37 | 38 | 39 | 40 | 41 | 42 | 43 | www.arduino.cc | 44 | 45 | 46 | 47 | TM | 48 | 49 | 50 | 51 | 52 | 53 | 0 | 1 | 2 | 3 | 4 | 5 | 6 | 7 | 8 | 9 | 10 | 11 | 12 | 13 | 14 | 15
tNames: SCL | SDA | M.Banzi | 5V | D.Cuartielles | T.Igoe | MADE IN | G.Martino | ITALY | D.Mellis | GND | AREF | PWM | TX | RX | TX3 | RX3 | TX2 | RX2 | TX1 | RX1 | SDA | SCL | 1 | DIGITAL | Arduino | MEGA 2560 | ANALOG IN | GND | IOREF | RESET | 3V3 | 5V | GND | VIN
bNames: MADE IN | designed by | ITALY | tinker it
ReferenceLC: L | ON | TX | RX | PC1 | PC2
